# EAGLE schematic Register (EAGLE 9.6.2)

## Sheet 1 of 3: adressen
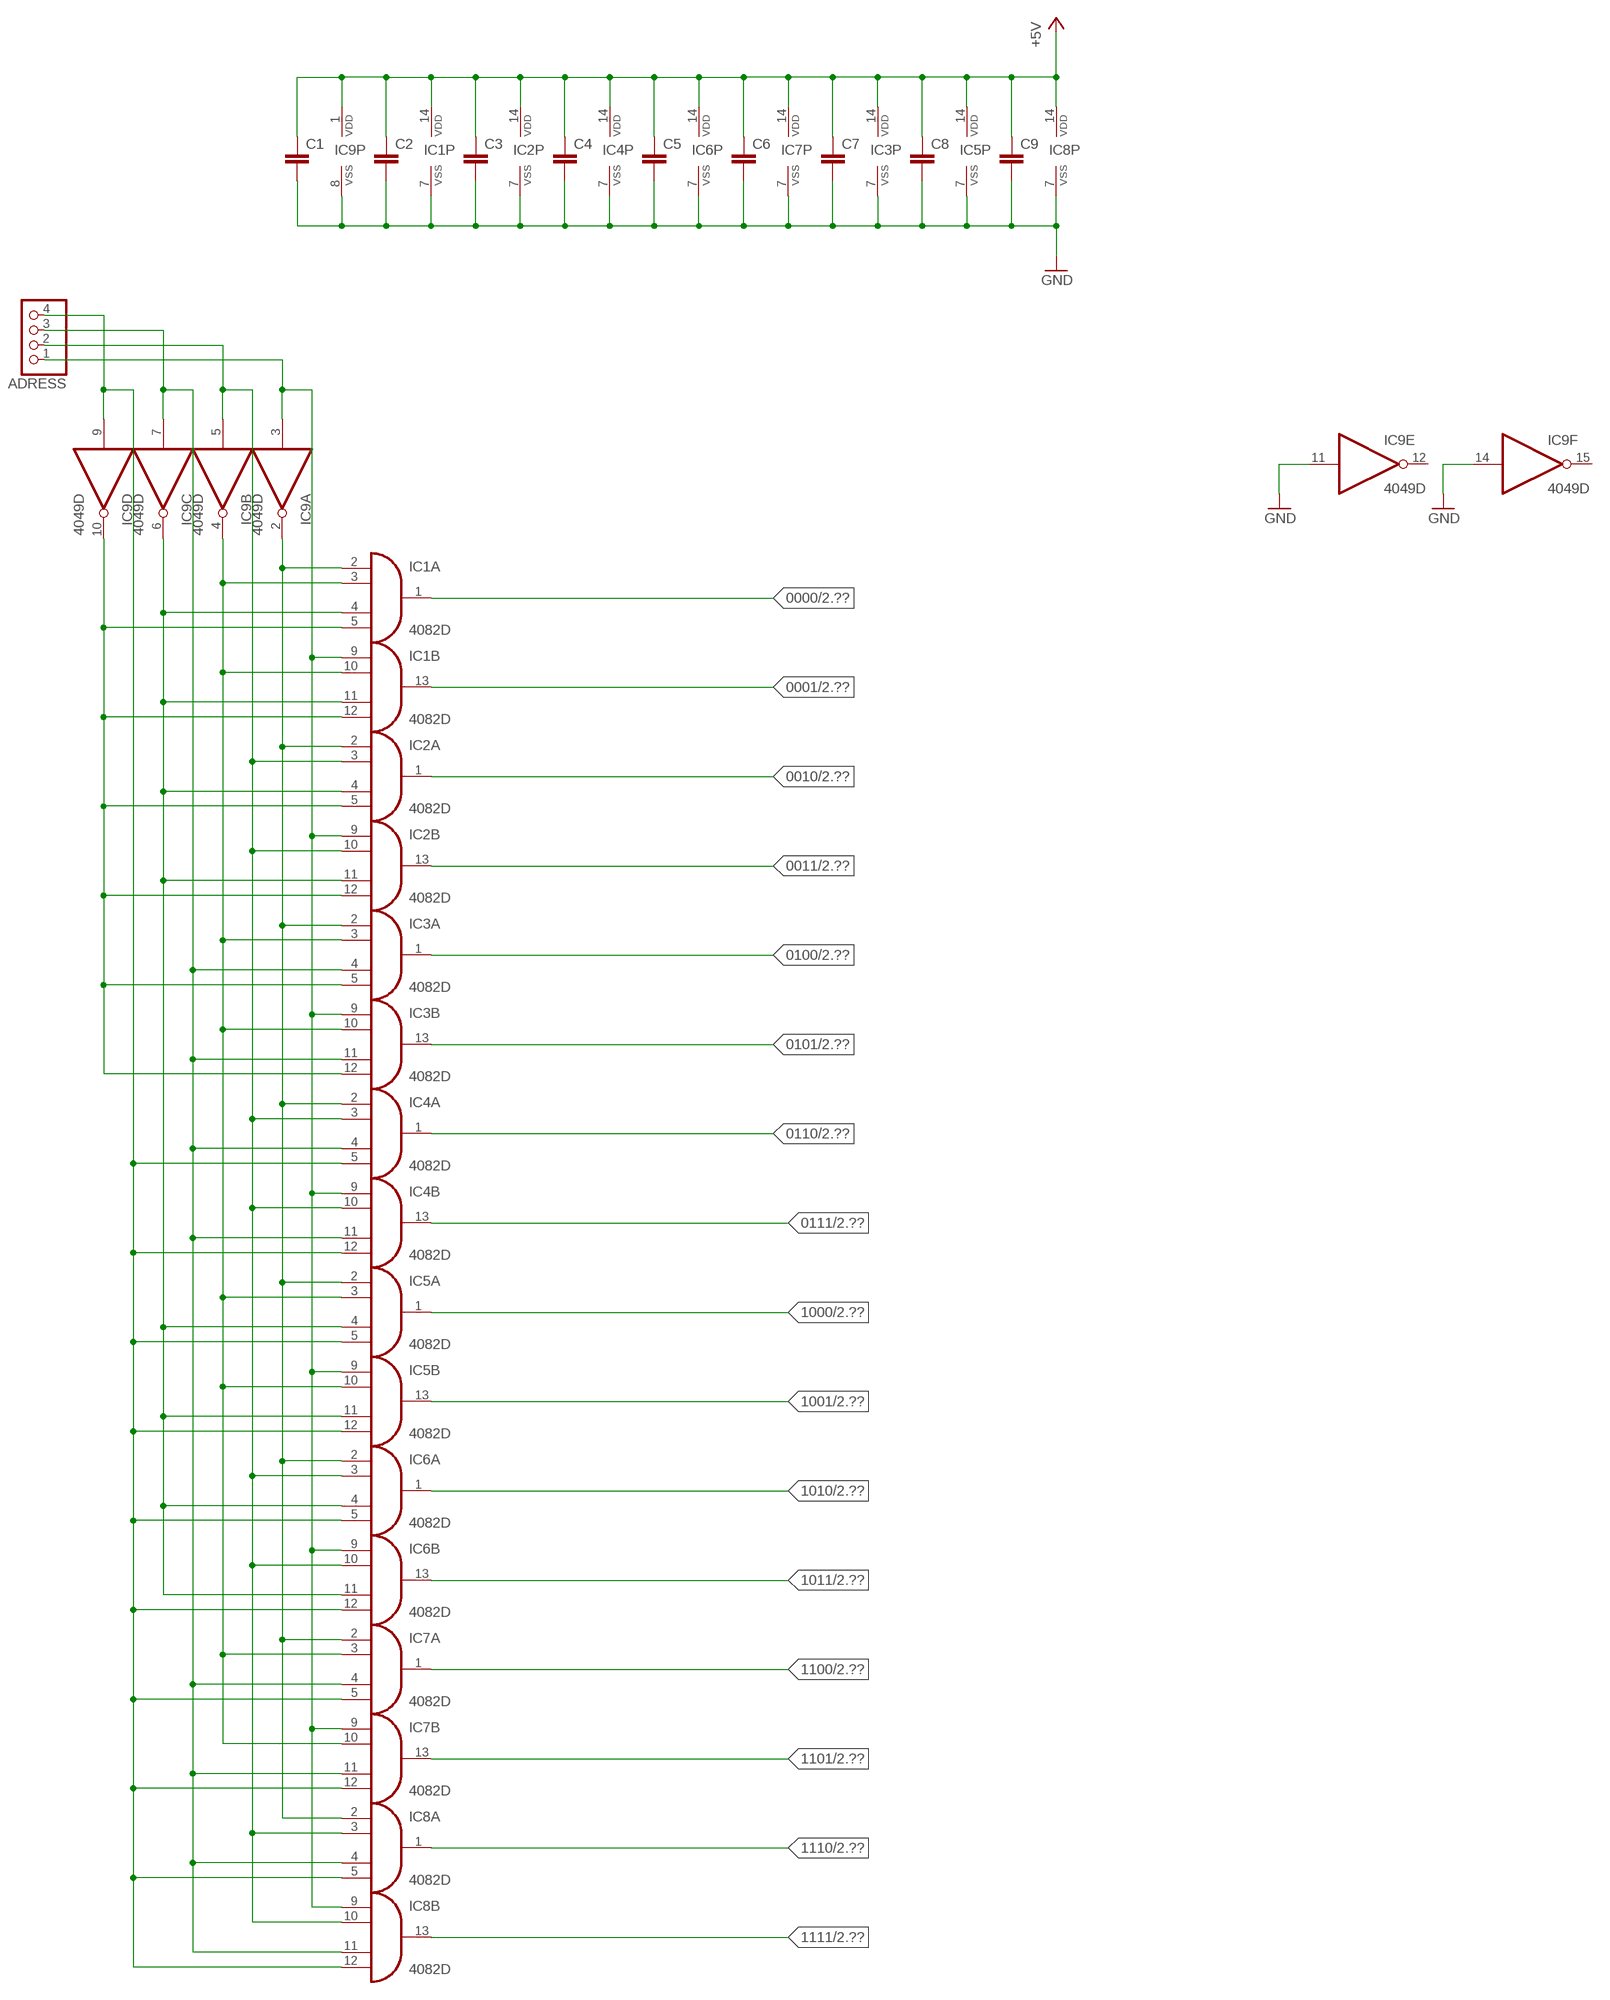
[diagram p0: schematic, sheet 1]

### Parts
ADRESS  PINHD-1X4  [1X04]
C1  C-EUC0805  [C0805]
C2  C-EUC0805  [C0805]
C3  C-EUC0805  [C0805]
C4  C-EUC0805  [C0805]
C5  C-EUC0805  [C0805]
C6  C-EUC0805  [C0805]
C7  C-EUC0805  [C0805]
C8  C-EUC0805  [C0805]
C9  C-EUC0805  [C0805]
IC1  4082D  [SO14]
IC2  4082D  [SO14]
IC3  4082D  [SO14]
IC4  4082D  [SO14]
IC5  4082D  [SO14]
IC6  4082D  [SO14]
IC7  4082D  [SO14]
IC8  4082D  [SO14]
IC9  4049D  [SO16]

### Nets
0000: IC1.1(A:O) ; also sheet 2
0001: IC1.13(B:O) ; also sheet 2
0010: IC2.1(A:O) ; also sheet 2
0011: IC2.13(B:O) ; also sheet 2
0100: IC3.1(A:O) ; also sheet 2
0101: IC3.13(B:O) ; also sheet 2
0110: IC4.1(A:O) ; also sheet 2
0111: IC4.13(B:O) ; also sheet 2
1000: IC5.1(A:O) ; also sheet 2
1001: IC5.13(B:O) ; also sheet 2
1010: IC6.1(A:O) ; also sheet 2
1011: IC6.13(B:O) ; also sheet 2
1100: IC7.1(A:O) ; also sheet 2
1101: IC7.13(B:O) ; also sheet 2
1110: IC8.1(A:O) ; also sheet 2
1111: IC8.13(B:O) ; also sheet 2
+5V: C1.1 C2.1 C3.1 C4.1 C5.1 C6.1 C7.1 C8.1 C9.1 IC1.14(P:VDD) IC2.14(P:VDD) IC3.14(P:VDD) IC4.14(P:VDD) IC5.14(P:VDD) IC6.14(P:VDD) IC7.14(P:VDD) IC8.14(P:VDD) IC9.1(P:VDD) ; also sheet 2,3
GND: C1.2 C2.2 C3.2 C4.2 C5.2 C6.2 C7.2 C8.2 C9.2 IC1.7(P:VSS) IC2.7(P:VSS) IC3.7(P:VSS) IC4.7(P:VSS) IC5.7(P:VSS) IC6.7(P:VSS) IC7.7(P:VSS) IC8.7(P:VSS) IC9.8(P:VSS) IC9.11(E:I) IC9.14(F:I) ; also sheet 2,3
N$1: ADRESS.1 IC1.9(B:I0) IC2.9(B:I0) IC3.9(B:I0) IC4.9(B:I0) IC5.9(B:I0) IC6.9(B:I0) IC7.9(B:I0) IC8.9(B:I0) IC9.3(A:I)
N$2: IC1.2(A:I0) IC2.2(A:I0) IC3.2(A:I0) IC4.2(A:I0) IC5.2(A:I0) IC6.2(A:I0) IC7.2(A:I0) IC8.2(A:I0) IC9.2(A:O)
N$3: ADRESS.2 IC2.3(A:I1) IC2.10(B:I1) IC4.3(A:I1) IC4.10(B:I1) IC6.3(A:I1) IC6.10(B:I1) IC8.3(A:I1) IC8.10(B:I1) IC9.5(B:I)
N$4: IC1.3(A:I1) IC1.10(B:I1) IC3.3(A:I1) IC3.10(B:I1) IC5.3(A:I1) IC5.10(B:I1) IC7.3(A:I1) IC7.10(B:I1) IC9.4(B:O)
N$5: ADRESS.3 IC3.4(A:I2) IC3.11(B:I2) IC4.4(A:I2) IC4.11(B:I2) IC7.4(A:I2) IC7.11(B:I2) IC8.4(A:I2) IC8.11(B:I2) IC9.7(C:I)
N$6: IC1.4(A:I2) IC1.11(B:I2) IC2.4(A:I2) IC2.11(B:I2) IC5.4(A:I2) IC5.11(B:I2) IC6.4(A:I2) IC6.11(B:I2) IC9.6(C:O)
N$7: ADRESS.4 IC4.5(A:I3) IC4.12(B:I3) IC5.5(A:I3) IC5.12(B:I3) IC6.5(A:I3) IC6.12(B:I3) IC7.5(A:I3) IC7.12(B:I3) IC8.5(A:I3) IC8.12(B:I3) IC9.9(D:I)
N$8: IC1.5(A:I3) IC1.12(B:I3) IC2.5(A:I3) IC2.12(B:I3) IC3.5(A:I3) IC3.12(B:I3) IC9.10(D:O)
Unconnected: IC9.12(E:O) IC9.15(F:O)

## Sheet 2 of 3: 4x4Speicher
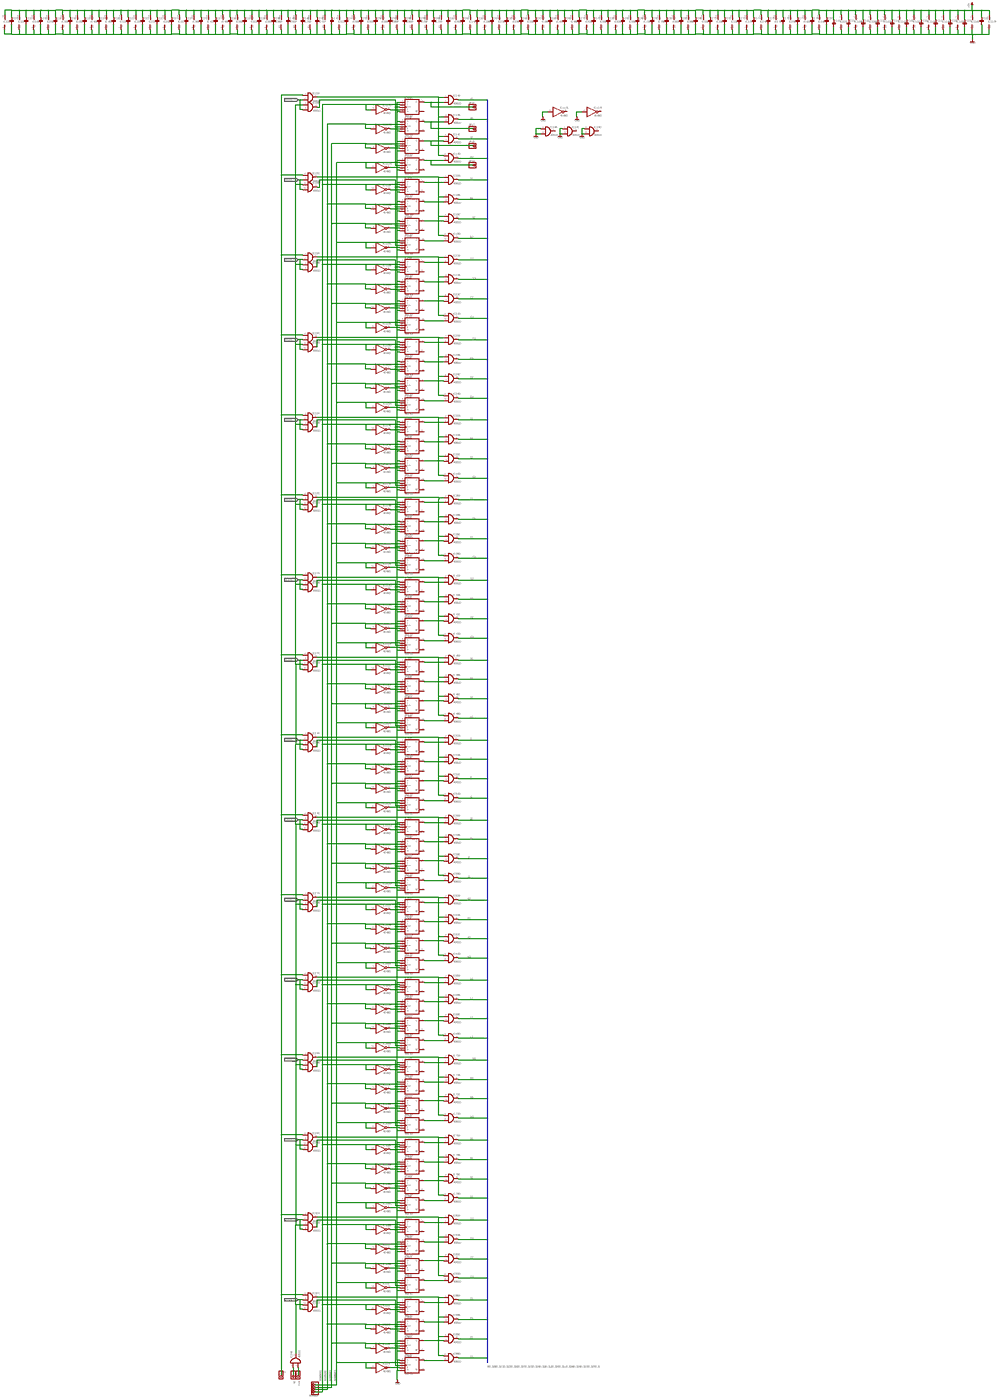
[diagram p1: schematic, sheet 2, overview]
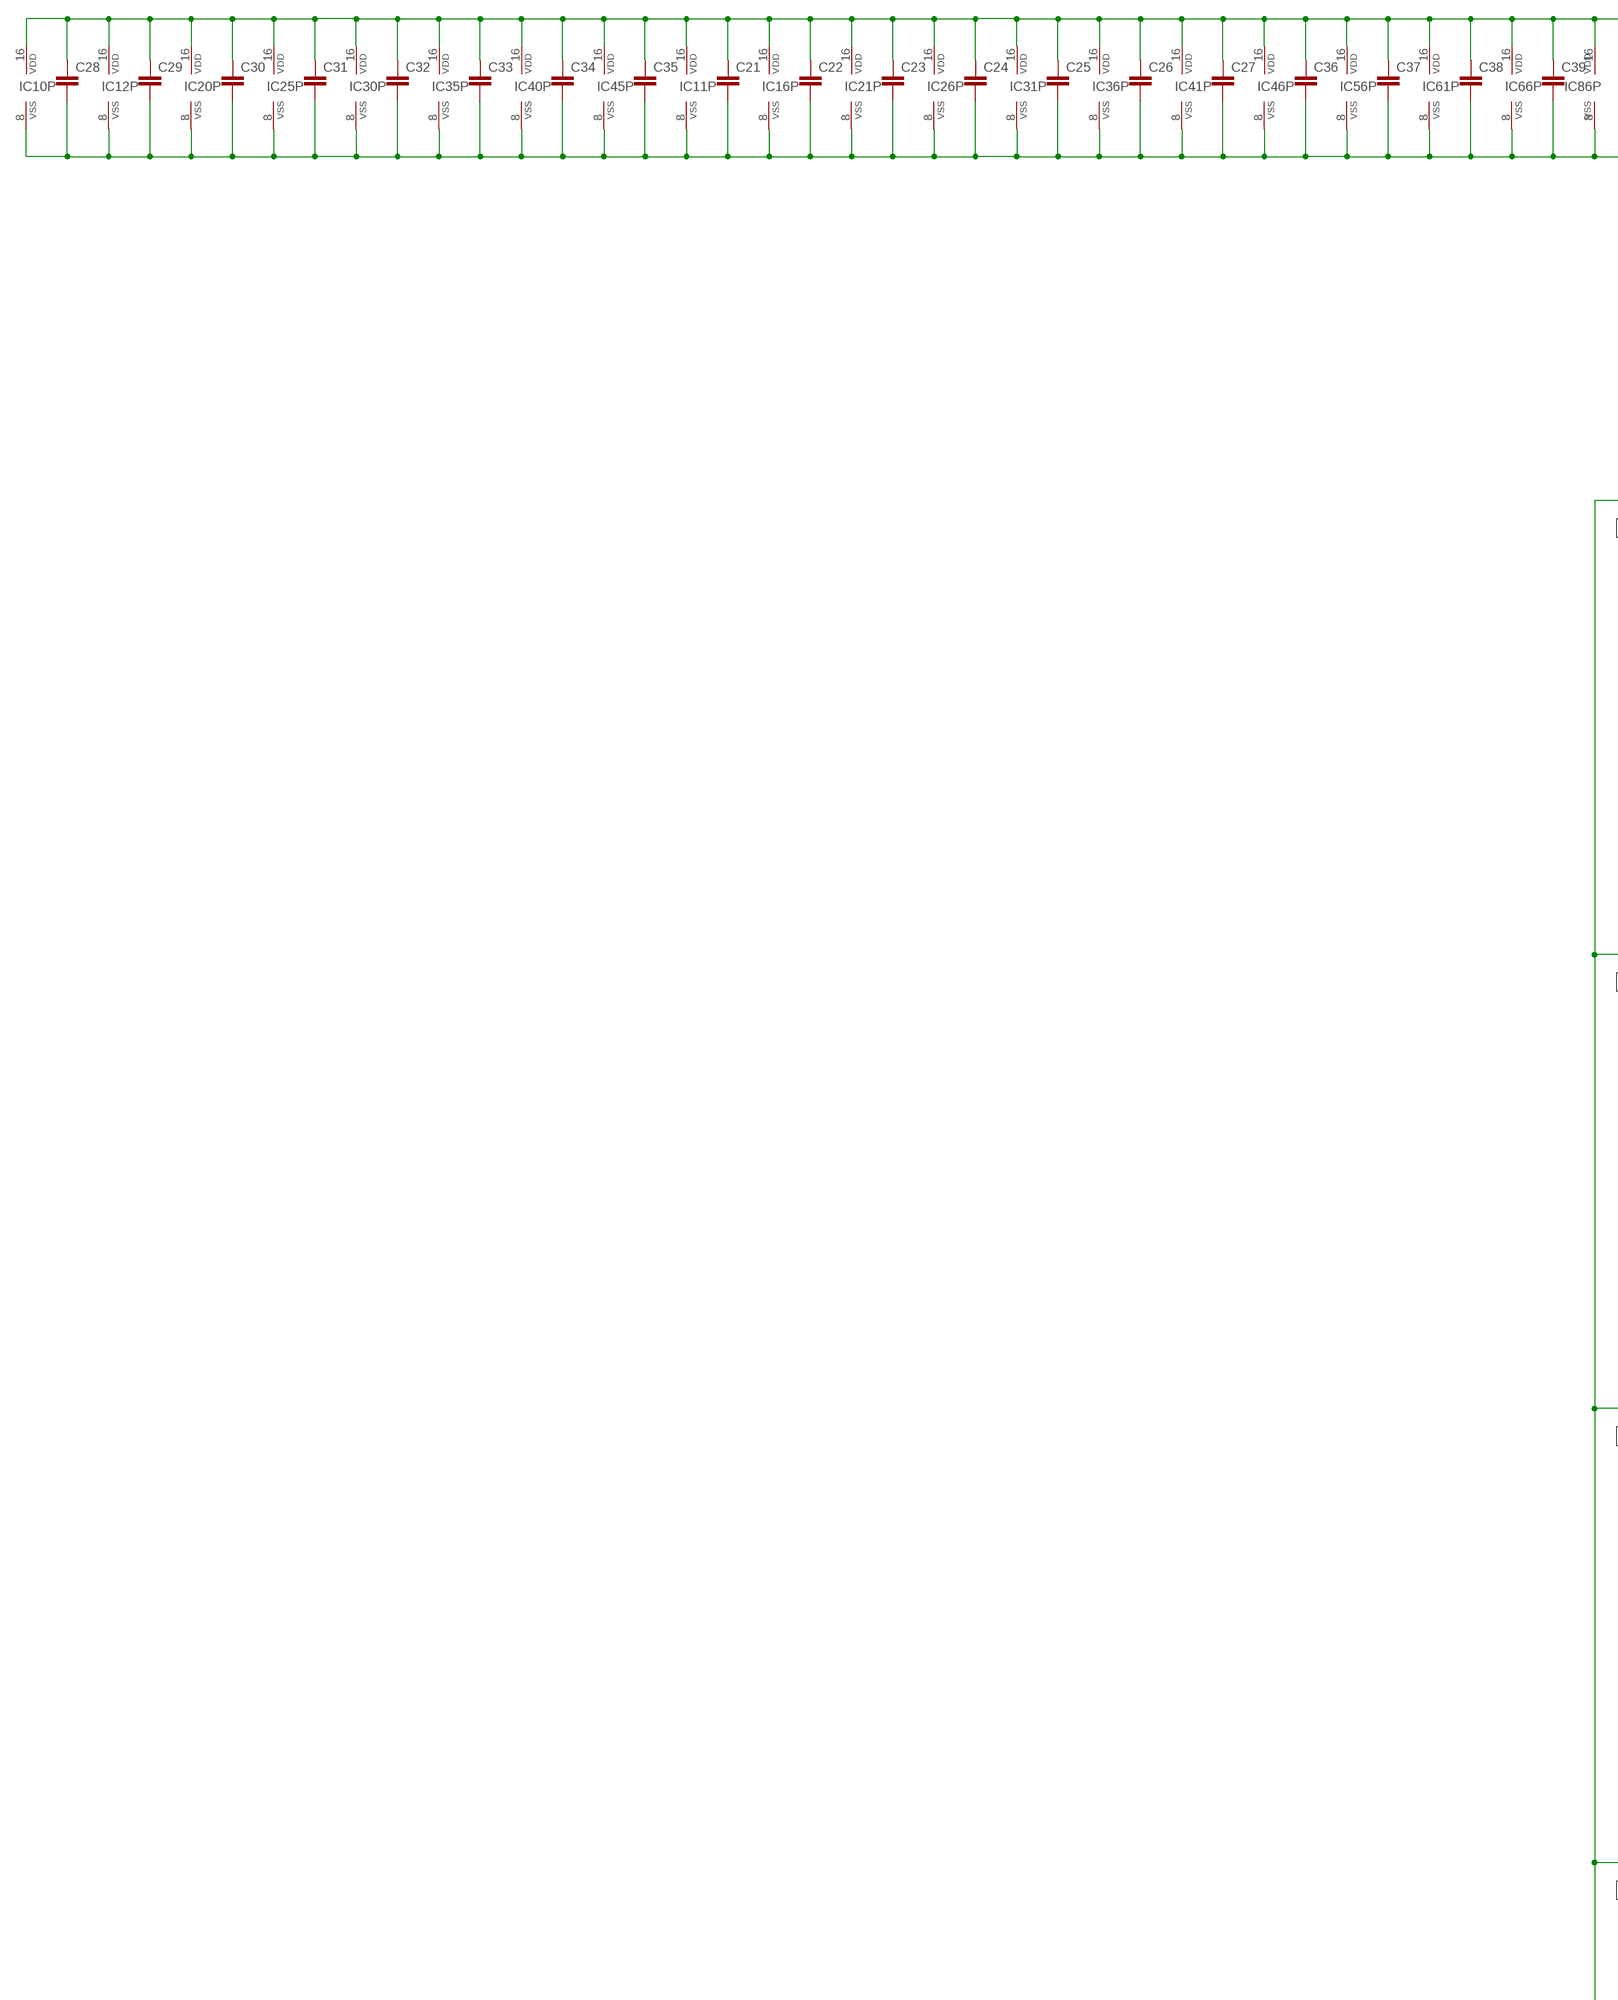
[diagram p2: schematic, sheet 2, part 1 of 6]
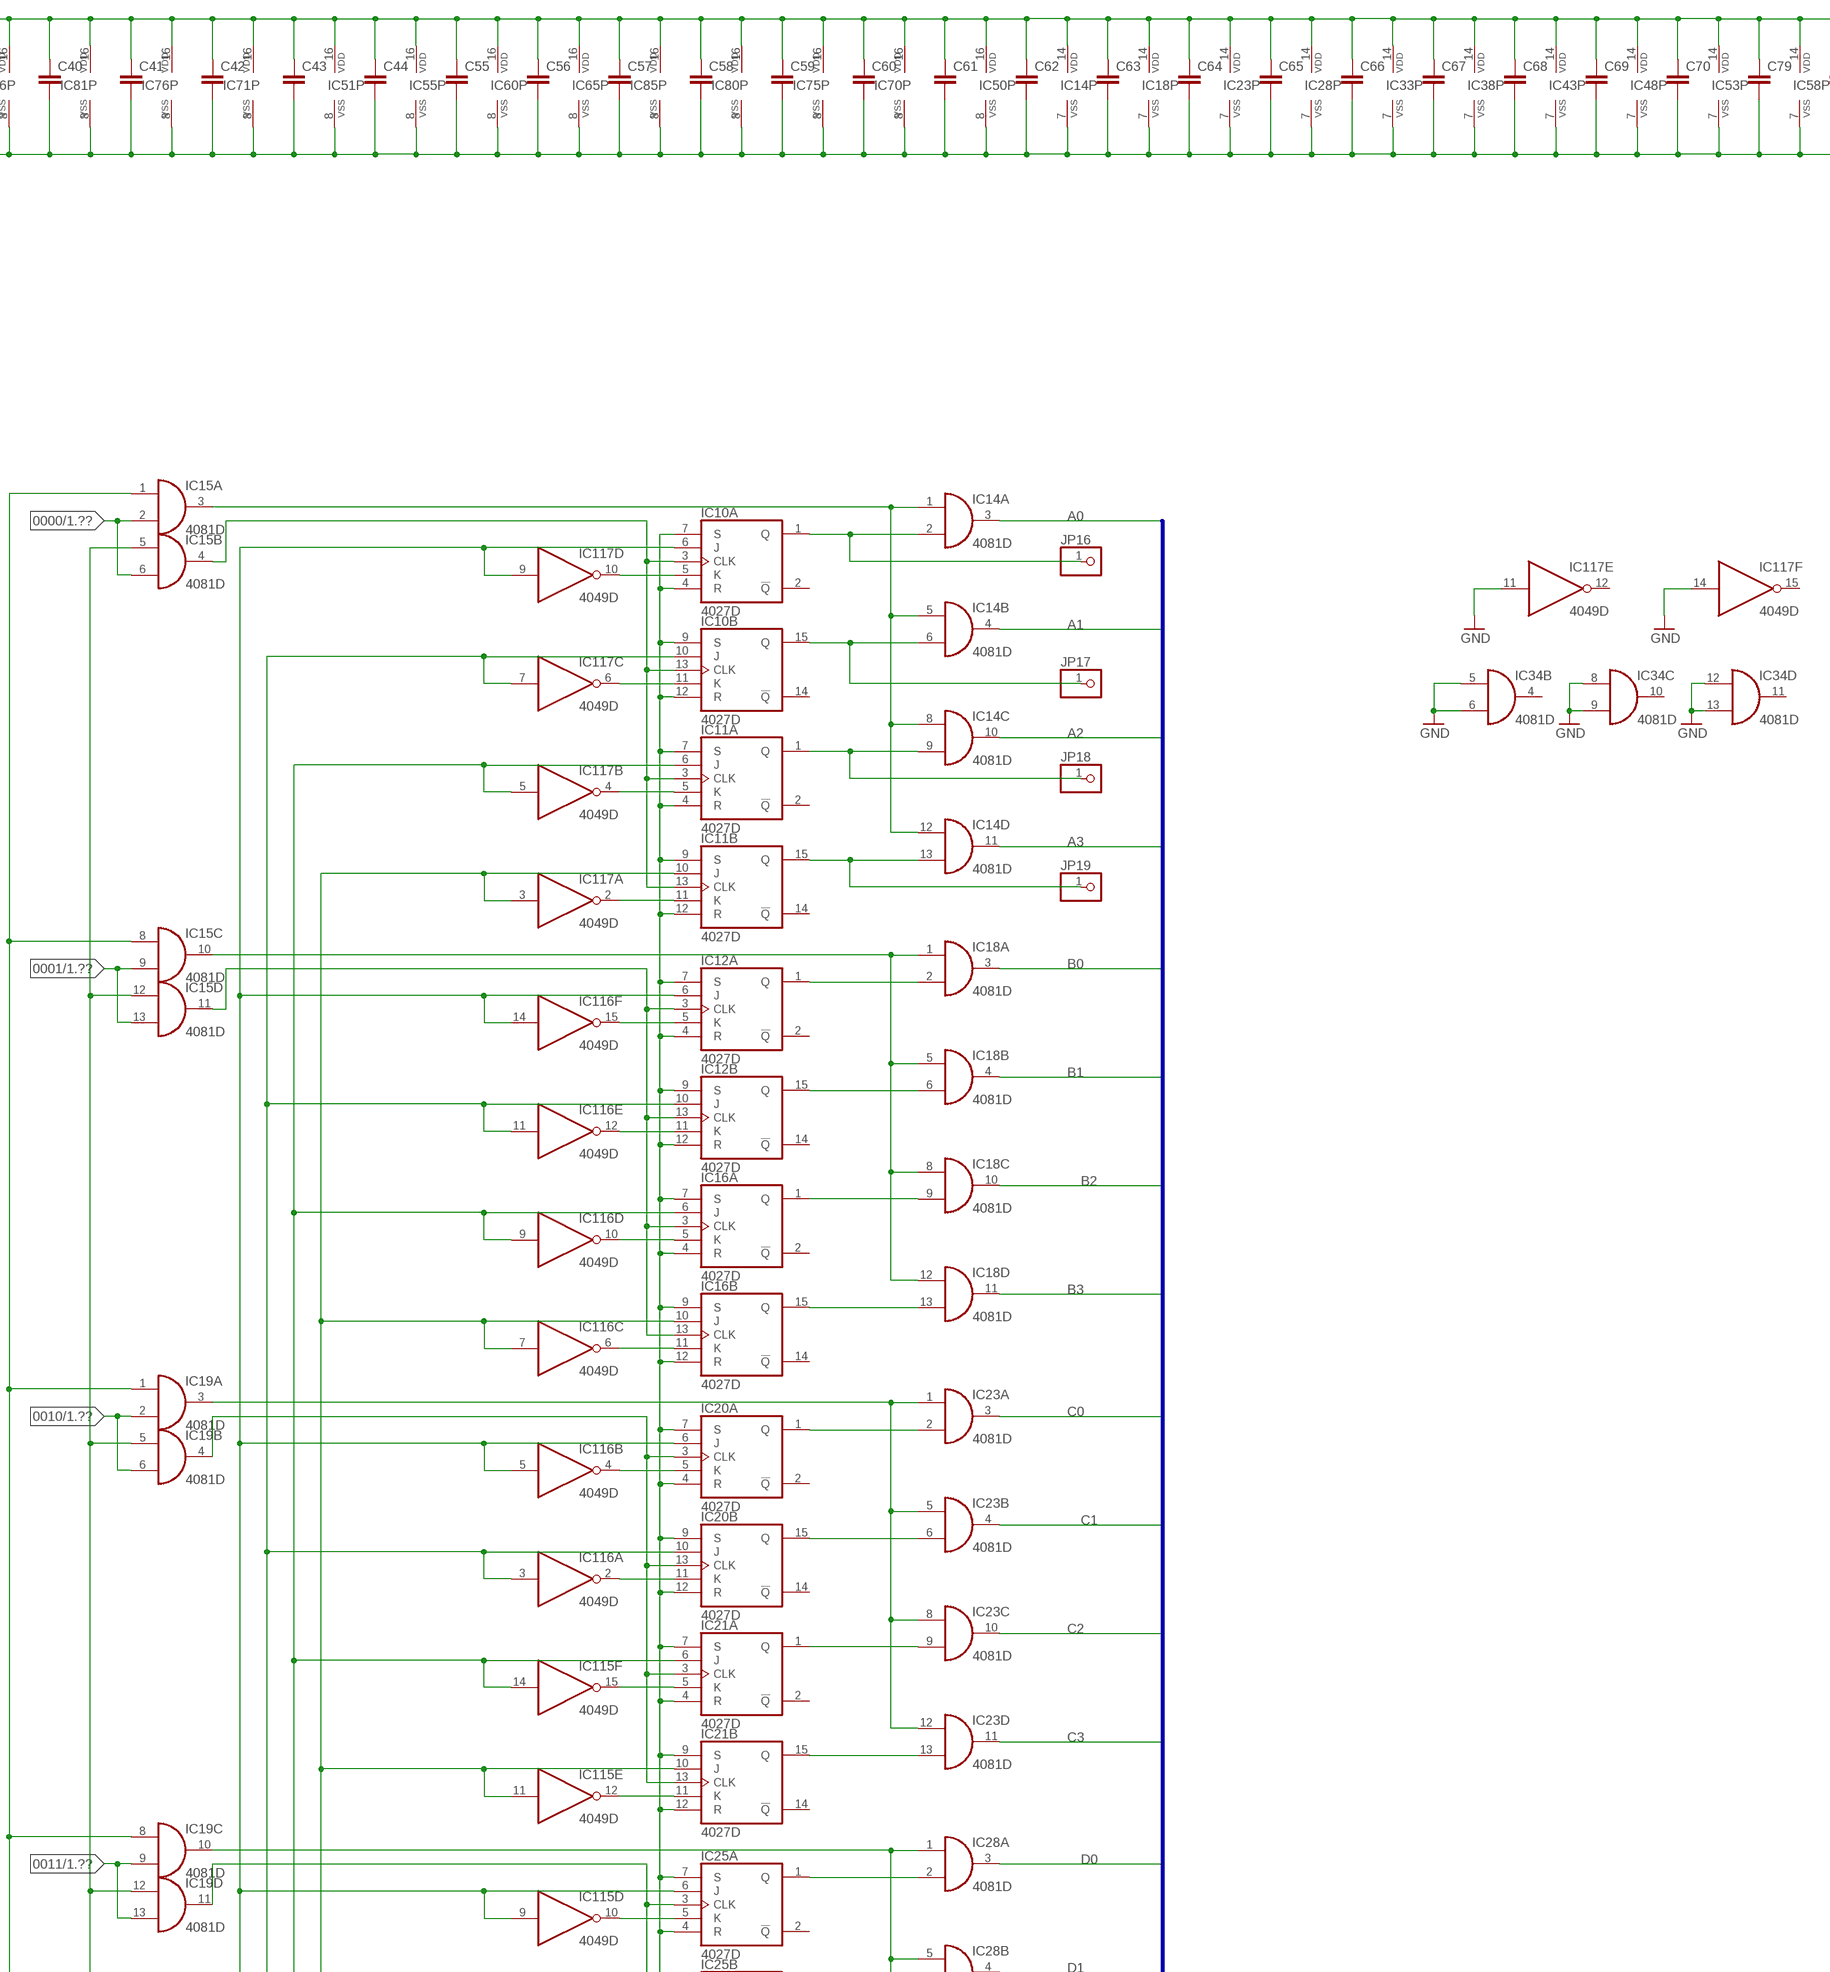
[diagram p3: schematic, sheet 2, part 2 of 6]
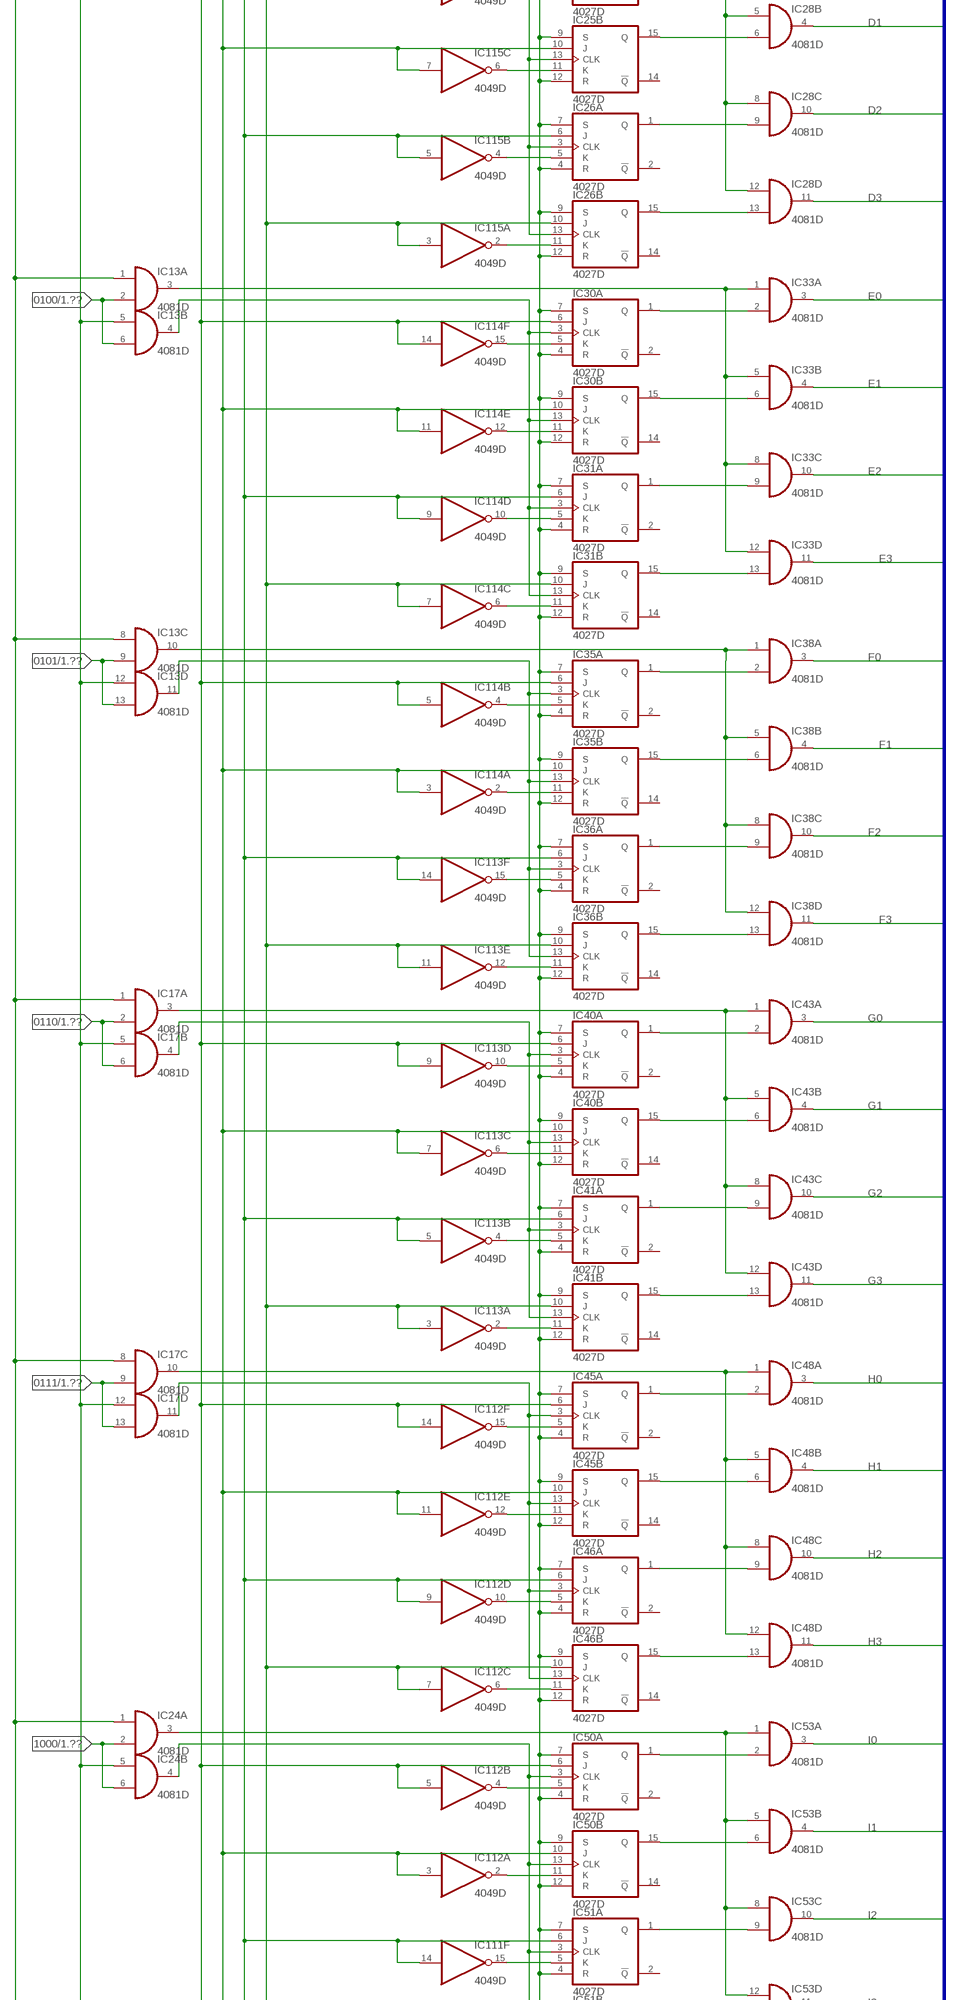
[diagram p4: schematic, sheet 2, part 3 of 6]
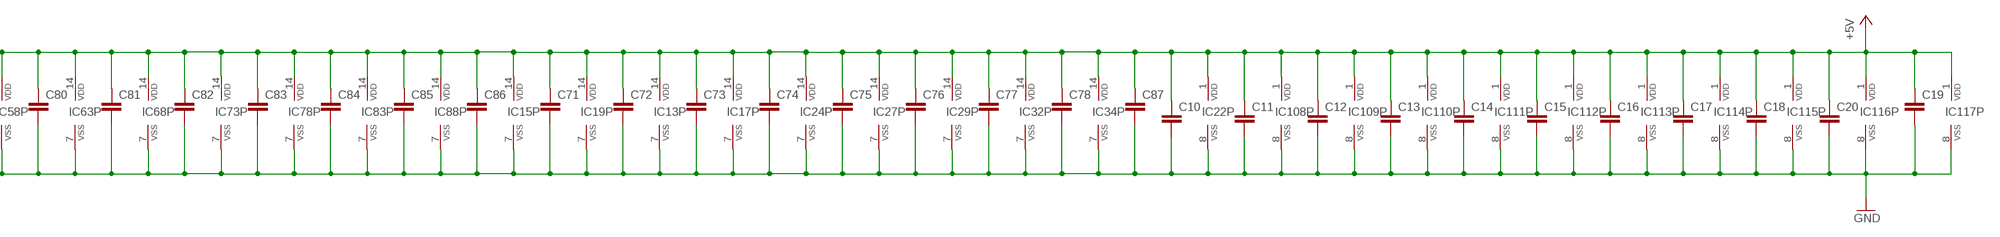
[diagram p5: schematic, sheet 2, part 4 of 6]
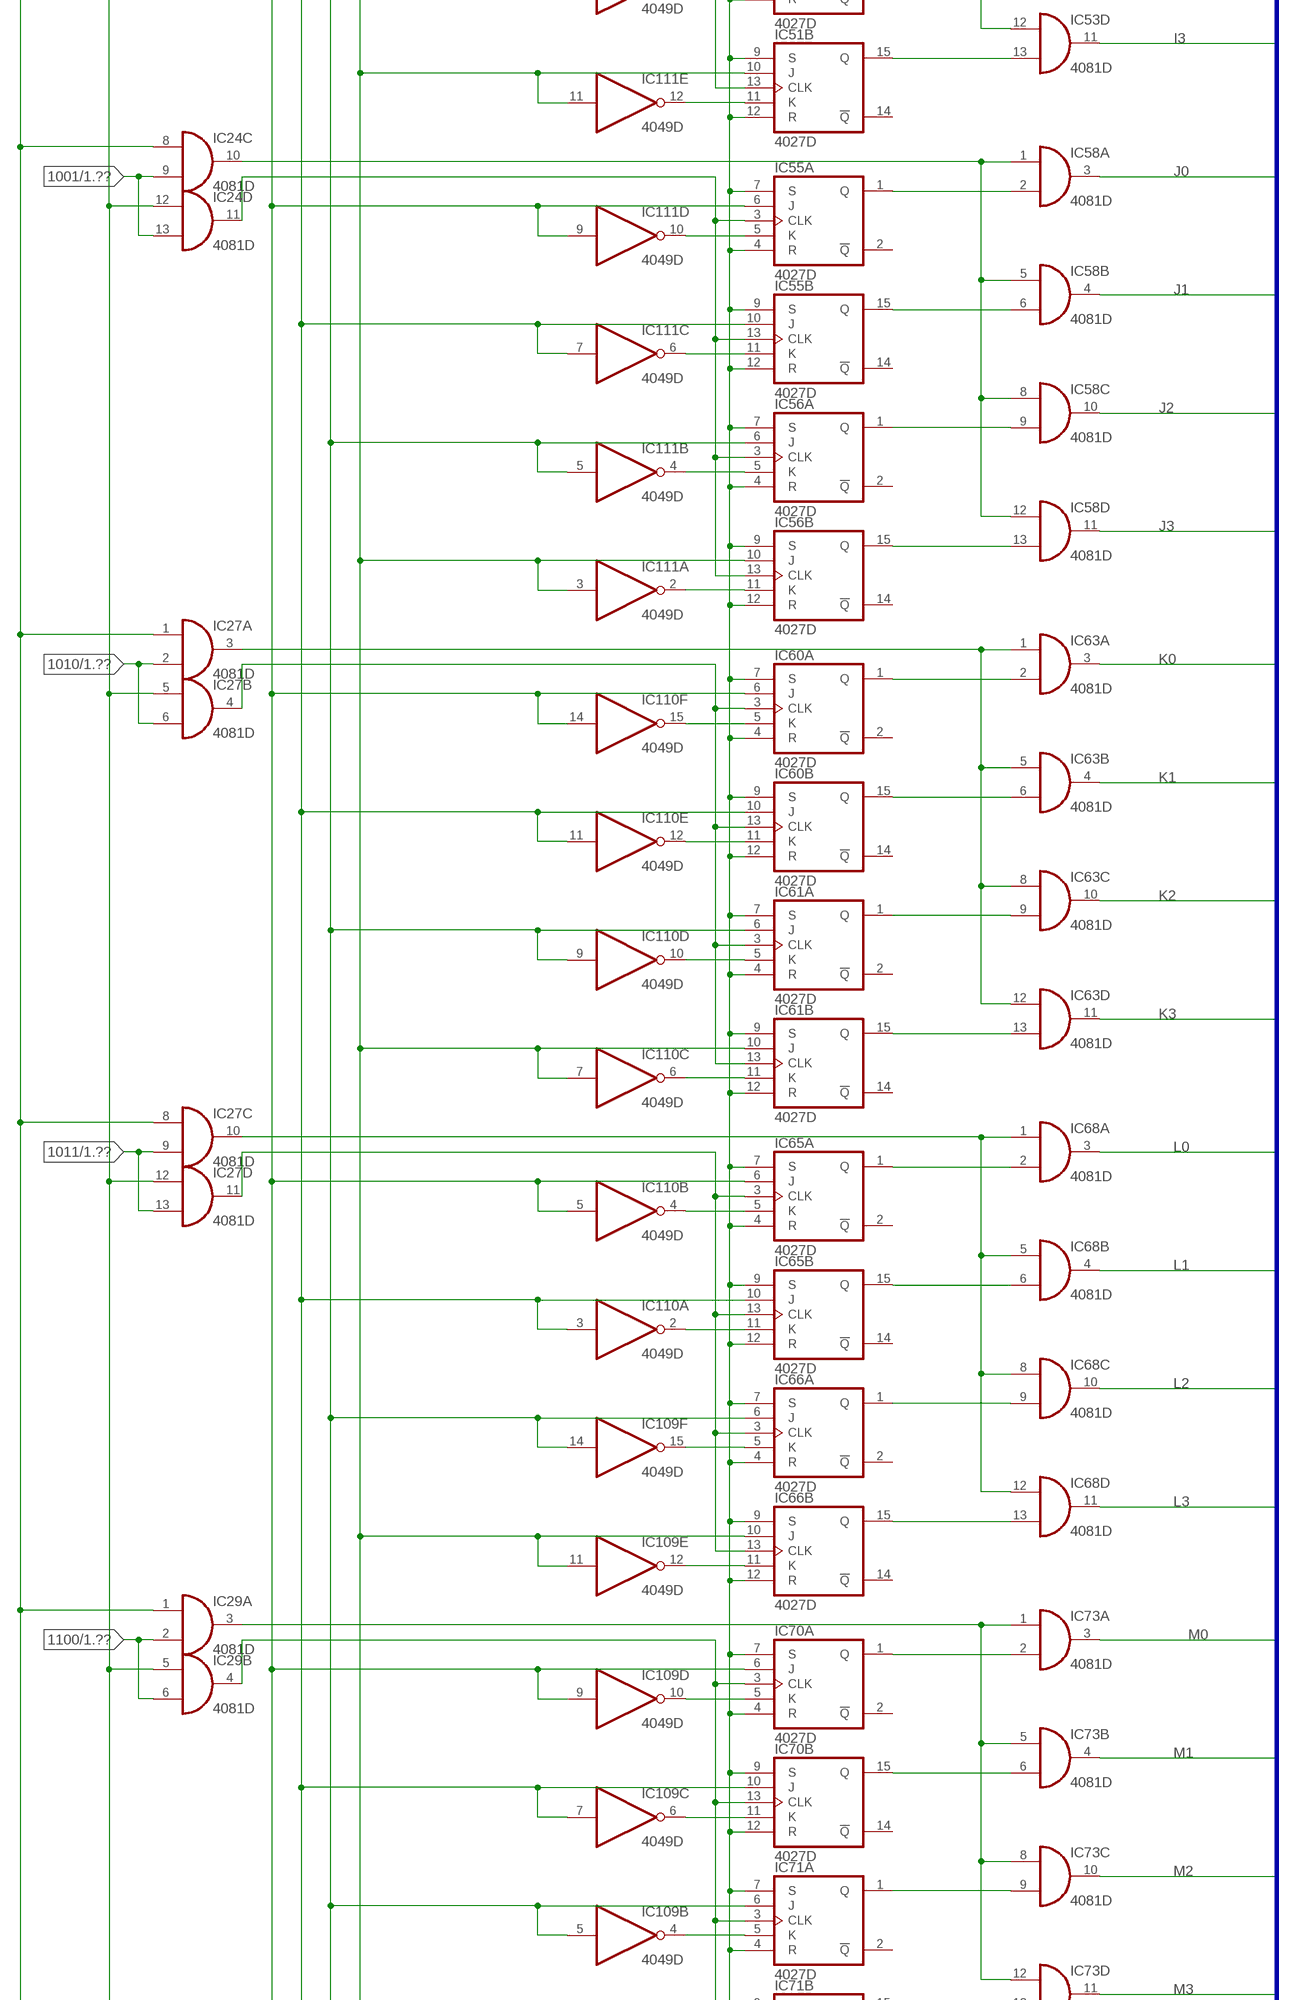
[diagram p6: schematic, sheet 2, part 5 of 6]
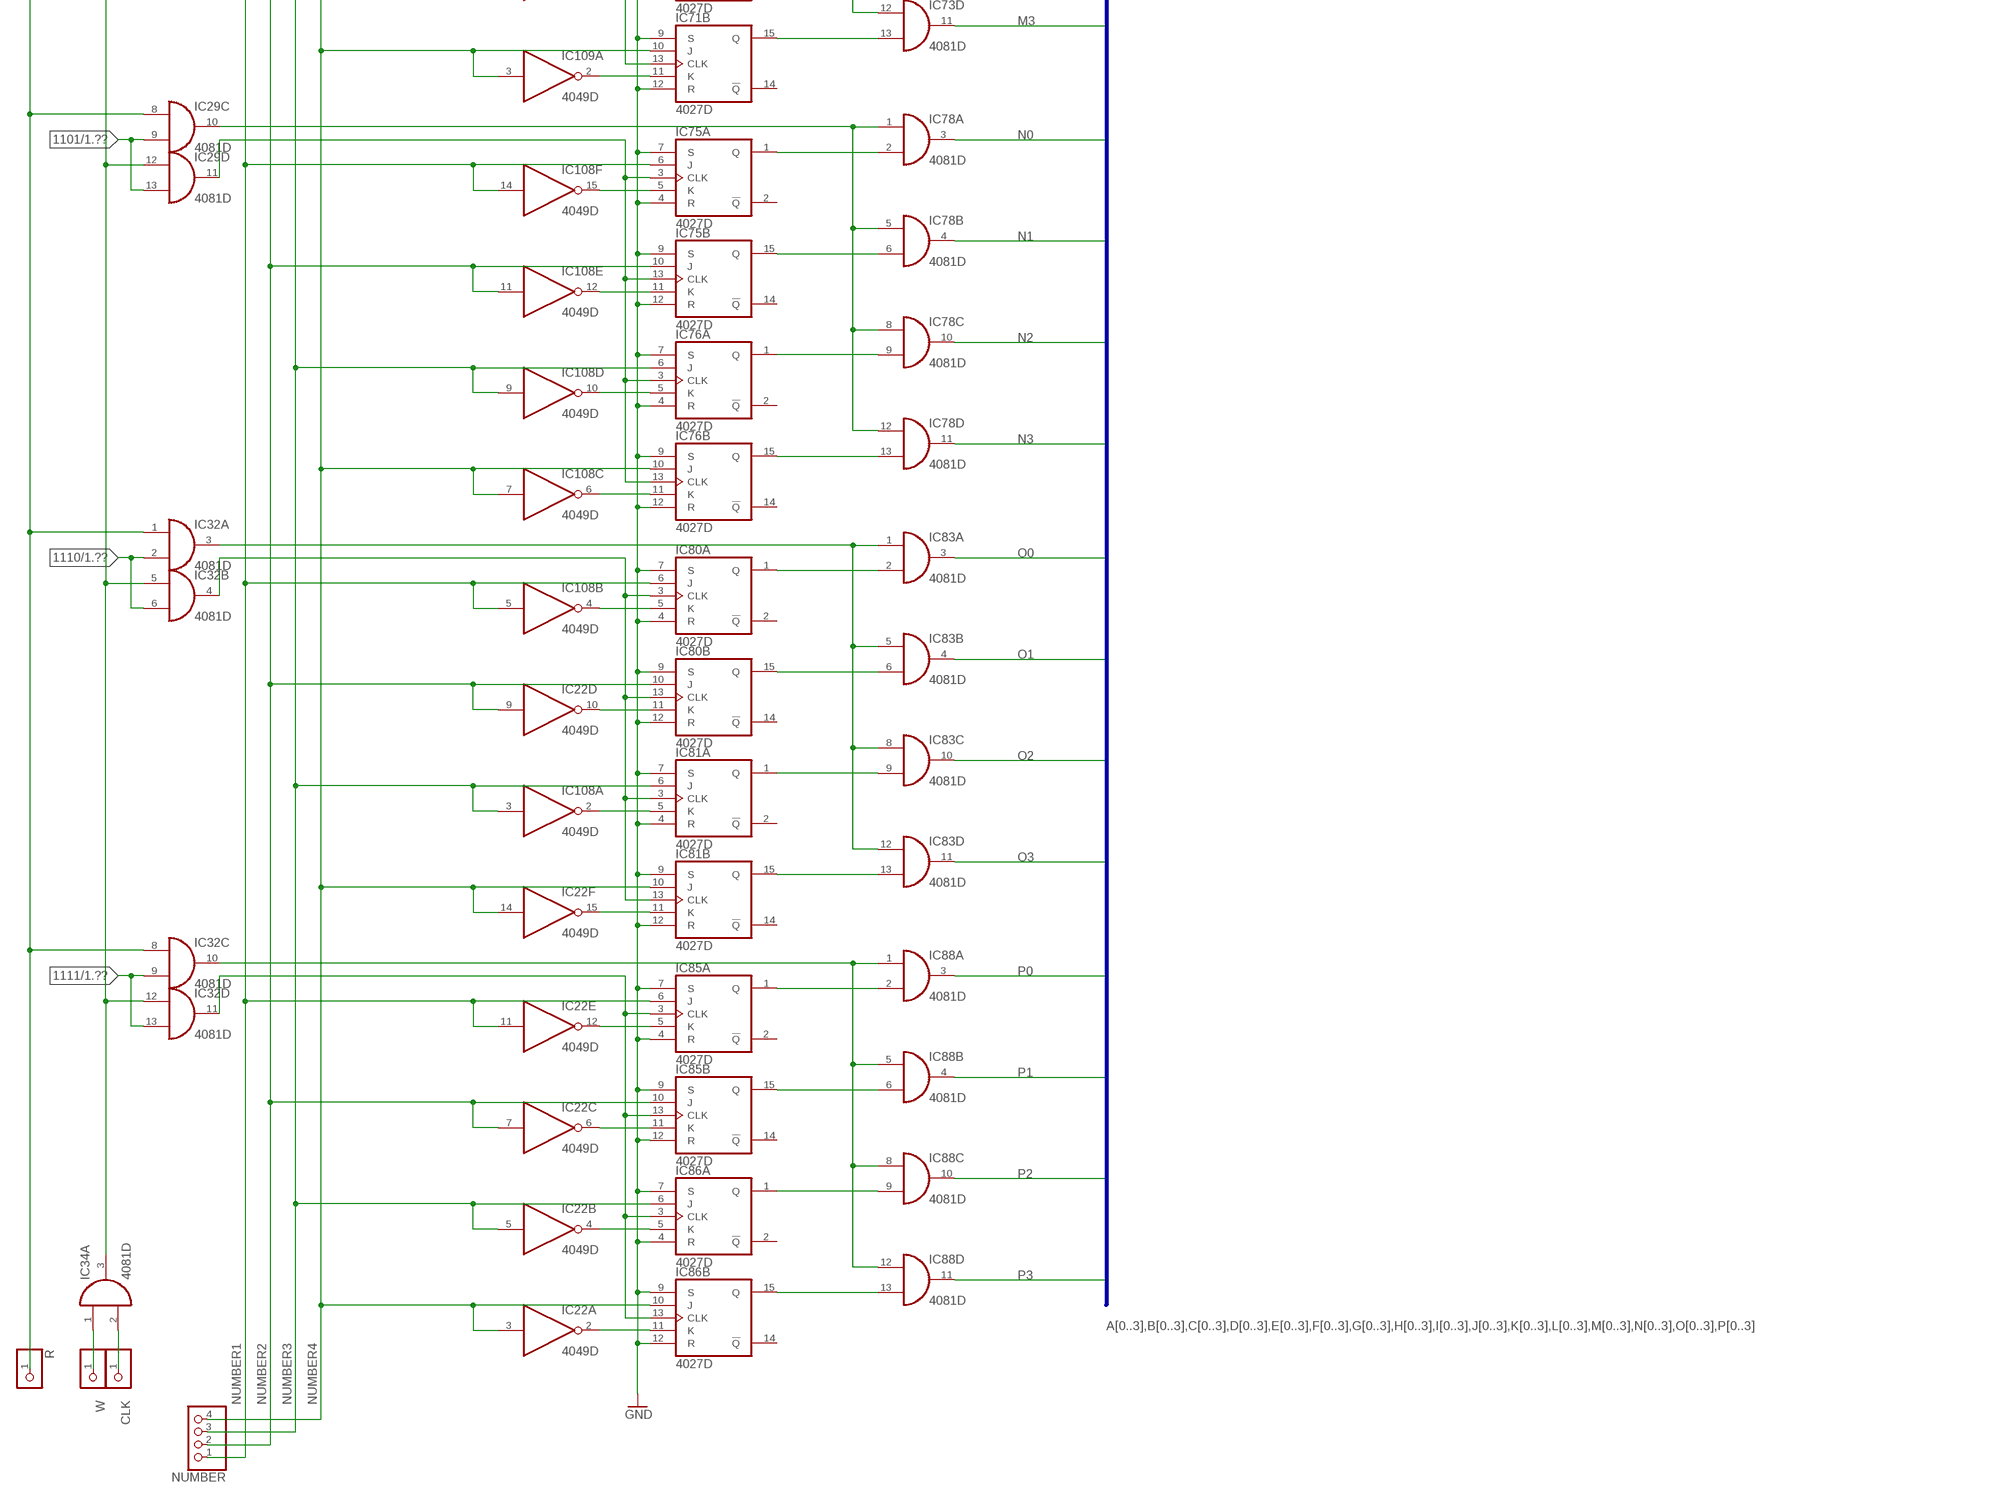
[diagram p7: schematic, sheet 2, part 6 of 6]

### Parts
C10  C-EUC0805  [C0805]
C11  C-EUC0805  [C0805]
C12  C-EUC0805  [C0805]
C13  C-EUC0805  [C0805]
C14  C-EUC0805  [C0805]
C15  C-EUC0805  [C0805]
C16  C-EUC0805  [C0805]
C17  C-EUC0805  [C0805]
C18  C-EUC0805  [C0805]
C19  C-EUC0805  [C0805]
C20  C-EUC0805  [C0805]
C21  C-EUC0805  [C0805]
C22  C-EUC0805  [C0805]
C23  C-EUC0805  [C0805]
C24  C-EUC0805  [C0805]
C25  C-EUC0805  [C0805]
C26  C-EUC0805  [C0805]
C27  C-EUC0805  [C0805]
C28  C-EUC0805  [C0805]
C29  C-EUC0805  [C0805]
C30  C-EUC0805  [C0805]
C31  C-EUC0805  [C0805]
C32  C-EUC0805  [C0805]
C33  C-EUC0805  [C0805]
C34  C-EUC0805  [C0805]
C35  C-EUC0805  [C0805]
C36  C-EUC0805  [C0805]
C37  C-EUC0805  [C0805]
C38  C-EUC0805  [C0805]
C39  C-EUC0805  [C0805]
C40  C-EUC0805  [C0805]
C41  C-EUC0805  [C0805]
C42  C-EUC0805  [C0805]
C43  C-EUC0805  [C0805]
C44  C-EUC0805  [C0805]
C55  C-EUC0805  [C0805]
C56  C-EUC0805  [C0805]
C57  C-EUC0805  [C0805]
C58  C-EUC0805  [C0805]
C59  C-EUC0805  [C0805]
C60  C-EUC0805  [C0805]
C61  C-EUC0805  [C0805]
C62  C-EUC0805  [C0805]
C63  C-EUC0805  [C0805]
C64  C-EUC0805  [C0805]
C65  C-EUC0805  [C0805]
C66  C-EUC0805  [C0805]
C67  C-EUC0805  [C0805]
C68  C-EUC0805  [C0805]
C69  C-EUC0805  [C0805]
C70  C-EUC0805  [C0805]
C71  C-EUC0805  [C0805]
C72  C-EUC0805  [C0805]
C73  C-EUC0805  [C0805]
C74  C-EUC0805  [C0805]
C75  C-EUC0805  [C0805]
C76  C-EUC0805  [C0805]
C77  C-EUC0805  [C0805]
C78  C-EUC0805  [C0805]
C79  C-EUC0805  [C0805]
C80  C-EUC0805  [C0805]
C81  C-EUC0805  [C0805]
C82  C-EUC0805  [C0805]
C83  C-EUC0805  [C0805]
C84  C-EUC0805  [C0805]
C85  C-EUC0805  [C0805]
C86  C-EUC0805  [C0805]
C87  C-EUC0805  [C0805]
CLK  PINHD-1X1  [1X01]
IC10  4027D  [SO16]
IC11  4027D  [SO16]
IC12  4027D  [SO16]
IC13  4081D  [SO14]
IC14  4081D  [SO14]
IC15  4081D  [SO14]
IC16  4027D  [SO16]
IC17  4081D  [SO14]
IC18  4081D  [SO14]
IC19  4081D  [SO14]
IC20  4027D  [SO16]
IC21  4027D  [SO16]
IC22  4049D  [SO16]
IC23  4081D  [SO14]
IC24  4081D  [SO14]
IC25  4027D  [SO16]
IC26  4027D  [SO16]
IC27  4081D  [SO14]
IC28  4081D  [SO14]
IC29  4081D  [SO14]
IC30  4027D  [SO16]
IC31  4027D  [SO16]
IC32  4081D  [SO14]
IC33  4081D  [SO14]
IC34  4081D  [SO14]
IC35  4027D  [SO16]
IC36  4027D  [SO16]
IC38  4081D  [SO14]
IC40  4027D  [SO16]
IC41  4027D  [SO16]
IC43  4081D  [SO14]
IC45  4027D  [SO16]
IC46  4027D  [SO16]
IC48  4081D  [SO14]
IC50  4027D  [SO16]
IC51  4027D  [SO16]
IC53  4081D  [SO14]
IC55  4027D  [SO16]
IC56  4027D  [SO16]
IC58  4081D  [SO14]
IC60  4027D  [SO16]
IC61  4027D  [SO16]
IC63  4081D  [SO14]
IC65  4027D  [SO16]
IC66  4027D  [SO16]
IC68  4081D  [SO14]
IC70  4027D  [SO16]
IC71  4027D  [SO16]
IC73  4081D  [SO14]
IC75  4027D  [SO16]
IC76  4027D  [SO16]
IC78  4081D  [SO14]
IC80  4027D  [SO16]
IC81  4027D  [SO16]
IC83  4081D  [SO14]
IC85  4027D  [SO16]
IC86  4027D  [SO16]
IC88  4081D  [SO14]
IC108  4049D  [SO16]
IC109  4049D  [SO16]
IC110  4049D  [SO16]
IC111  4049D  [SO16]
IC112  4049D  [SO16]
IC113  4049D  [SO16]
IC114  4049D  [SO16]
IC115  4049D  [SO16]
IC116  4049D  [SO16]
IC117  4049D  [SO16]
JP16  PINHD-1X1  [1X01]
JP17  PINHD-1X1  [1X01]
JP18  PINHD-1X1  [1X01]
JP19  PINHD-1X1  [1X01]
NUMBER  PINHD-1X4  [1X04]
R  PINHD-1X1  [1X01]
W  PINHD-1X1  [1X01]

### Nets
0000: IC15.2(A:I1) IC15.6(B:I1) ; also sheet 1
0001: IC15.9(C:I1) IC15.13(D:I1) ; also sheet 1
0010: IC19.2(A:I1) IC19.6(B:I1) ; also sheet 1
0011: IC19.9(C:I1) IC19.13(D:I1) ; also sheet 1
0100: IC13.2(A:I1) IC13.6(B:I1) ; also sheet 1
0101: IC13.9(C:I1) IC13.13(D:I1) ; also sheet 1
0110: IC17.2(A:I1) IC17.6(B:I1) ; also sheet 1
0111: IC17.9(C:I1) IC17.13(D:I1) ; also sheet 1
1000: IC24.2(A:I1) IC24.6(B:I1) ; also sheet 1
1001: IC24.9(C:I1) IC24.13(D:I1) ; also sheet 1
1010: IC27.2(A:I1) IC27.6(B:I1) ; also sheet 1
1011: IC27.9(C:I1) IC27.13(D:I1) ; also sheet 1
1100: IC29.2(A:I1) IC29.6(B:I1) ; also sheet 1
1101: IC29.9(C:I1) IC29.13(D:I1) ; also sheet 1
1110: IC32.2(A:I1) IC32.6(B:I1) ; also sheet 1
1111: IC32.9(C:I1) IC32.13(D:I1) ; also sheet 1
+5V: C10.1 C11.1 C12.1 C13.1 C14.1 C15.1 C16.1 C17.1 C18.1 C19.1 C20.1 C21.1 C22.1 C23.1 C24.1 C25.1 C26.1 C27.1 C28.1 C29.1 C30.1 C31.1 C32.1 C33.1 C34.1 C35.1 C36.1 C37.1 C38.1 C39.1 C40.1 C41.1 C42.1 C43.1 C44.1 C55.1 C56.1 C57.1 C58.1 C59.1 C60.1 C61.1 C62.1 C63.1 C64.1 C65.1 C66.1 C67.1 C68.1 C69.1 C70.1 C71.1 C72.1 C73.1 C74.1 C75.1 C76.1 C77.1 C78.1 C79.1 C80.1 C81.1 C82.1 C83.1 C84.1 C85.1 C86.1 C87.1 IC10.16(P:VDD) IC11.16(P:VDD) IC12.16(P:VDD) IC13.14(P:VDD) IC14.14(P:VDD) IC15.14(P:VDD) IC16.16(P:VDD) IC17.14(P:VDD) IC18.14(P:VDD) IC19.14(P:VDD) IC20.16(P:VDD) IC21.16(P:VDD) IC22.1(P:VDD) IC23.14(P:VDD) IC24.14(P:VDD) IC25.16(P:VDD) IC26.16(P:VDD) IC27.14(P:VDD) IC28.14(P:VDD) IC29.14(P:VDD) IC30.16(P:VDD) IC31.16(P:VDD) IC32.14(P:VDD) IC33.14(P:VDD) IC34.14(P:VDD) IC35.16(P:VDD) IC36.16(P:VDD) IC38.14(P:VDD) IC40.16(P:VDD) IC41.16(P:VDD) IC43.14(P:VDD) IC45.16(P:VDD) IC46.16(P:VDD) IC48.14(P:VDD) IC50.16(P:VDD) IC51.16(P:VDD) IC53.14(P:VDD) IC55.16(P:VDD) IC56.16(P:VDD) IC58.14(P:VDD) IC60.16(P:VDD) IC61.16(P:VDD) IC63.14(P:VDD) IC65.16(P:VDD) IC66.16(P:VDD) IC68.14(P:VDD) IC70.16(P:VDD) IC71.16(P:VDD) IC73.14(P:VDD) IC75.16(P:VDD) IC76.16(P:VDD) IC78.14(P:VDD) IC80.16(P:VDD) IC81.16(P:VDD) IC83.14(P:VDD) IC85.16(P:VDD) IC86.16(P:VDD) IC88.14(P:VDD) IC108.1(P:VDD) IC109.1(P:VDD) IC110.1(P:VDD) IC111.1(P:VDD) IC112.1(P:VDD) IC113.1(P:VDD) IC114.1(P:VDD) IC115.1(P:VDD) IC116.1(P:VDD) IC117.1(P:VDD) ; also sheet 1,3
A0: IC14.3(A:O) ; also sheet 3
A1: IC14.4(B:O) ; also sheet 3
A2: IC14.10(C:O) ; also sheet 3
A3: IC14.11(D:O) ; also sheet 3
B0: IC18.3(A:O) ; also sheet 3
B1: IC18.4(B:O) ; also sheet 3
B2: IC18.10(C:O) ; also sheet 3
B3: IC18.11(D:O) ; also sheet 3
C0: IC23.3(A:O) ; also sheet 3
C1: IC23.4(B:O) ; also sheet 3
C2: IC23.10(C:O) ; also sheet 3
C3: IC23.11(D:O) ; also sheet 3
D0: IC28.3(A:O) ; also sheet 3
D1: IC28.4(B:O) ; also sheet 3
D2: IC28.10(C:O) ; also sheet 3
D3: IC28.11(D:O) ; also sheet 3
E0: IC33.3(A:O) ; also sheet 3
E1: IC33.4(B:O) ; also sheet 3
E2: IC33.10(C:O) ; also sheet 3
E3: IC33.11(D:O) ; also sheet 3
F0: IC38.3(A:O) ; also sheet 3
F1: IC38.4(B:O) ; also sheet 3
F2: IC38.10(C:O) ; also sheet 3
F3: IC38.11(D:O) ; also sheet 3
G0: IC43.3(A:O) ; also sheet 3
G1: IC43.4(B:O) ; also sheet 3
G2: IC43.10(C:O) ; also sheet 3
G3: IC43.11(D:O) ; also sheet 3
GND: C10.2 C11.2 C12.2 C13.2 C14.2 C15.2 C16.2 C17.2 C18.2 C19.2 C20.2 C21.2 C22.2 C23.2 C24.2 C25.2 C26.2 C27.2 C28.2 C29.2 C30.2 C31.2 C32.2 C33.2 C34.2 C35.2 C36.2 C37.2 C38.2 C39.2 C40.2 C41.2 C42.2 C43.2 C44.2 C55.2 C56.2 C57.2 C58.2 C59.2 C60.2 C61.2 C62.2 C63.2 C64.2 C65.2 C66.2 C67.2 C68.2 C69.2 C70.2 C71.2 C72.2 C73.2 C74.2 C75.2 C76.2 C77.2 C78.2 C79.2 C80.2 C81.2 C82.2 C83.2 C84.2 C85.2 C86.2 C87.2 IC10.4(A:R) IC10.7(A:S) IC10.8(P:VSS) IC10.9(B:S) IC10.12(B:R) IC11.4(A:R) IC11.7(A:S) IC11.8(P:VSS) IC11.9(B:S) IC11.12(B:R) IC12.4(A:R) IC12.7(A:S) IC12.8(P:VSS) IC12.9(B:S) IC12.12(B:R) IC13.7(P:VSS) IC14.7(P:VSS) IC15.7(P:VSS) IC16.4(A:R) IC16.7(A:S) IC16.8(P:VSS) IC16.9(B:S) IC16.12(B:R) IC17.7(P:VSS) IC18.7(P:VSS) IC19.7(P:VSS) IC20.4(A:R) IC20.7(A:S) IC20.8(P:VSS) IC20.9(B:S) IC20.12(B:R) IC21.4(A:R) IC21.7(A:S) IC21.8(P:VSS) IC21.9(B:S) IC21.12(B:R) IC22.8(P:VSS) IC23.7(P:VSS) IC24.7(P:VSS) IC25.4(A:R) IC25.7(A:S) IC25.8(P:VSS) IC25.9(B:S) IC25.12(B:R) IC26.4(A:R) IC26.7(A:S) IC26.8(P:VSS) IC26.9(B:S) IC26.12(B:R) IC27.7(P:VSS) IC28.7(P:VSS) IC29.7(P:VSS) IC30.4(A:R) IC30.7(A:S) IC30.8(P:VSS) IC30.9(B:S) IC30.12(B:R) IC31.4(A:R) IC31.7(A:S) IC31.8(P:VSS) IC31.9(B:S) IC31.12(B:R) IC32.7(P:VSS) IC33.7(P:VSS) IC34.5(B:I0) IC34.6(B:I1) IC34.7(P:VSS) IC34.8(C:I0) IC34.9(C:I1) IC34.12(D:I0) IC34.13(D:I1) IC35.4(A:R) IC35.7(A:S) IC35.8(P:VSS) IC35.9(B:S) IC35.12(B:R) IC36.4(A:R) IC36.7(A:S) IC36.8(P:VSS) IC36.9(B:S) IC36.12(B:R) IC38.7(P:VSS) IC40.4(A:R) IC40.7(A:S) IC40.8(P:VSS) IC40.9(B:S) IC40.12(B:R) IC41.4(A:R) IC41.7(A:S) IC41.8(P:VSS) IC41.9(B:S) IC41.12(B:R) IC43.7(P:VSS) IC45.4(A:R) IC45.7(A:S) IC45.8(P:VSS) IC45.9(B:S) IC45.12(B:R) IC46.4(A:R) IC46.7(A:S) IC46.8(P:VSS) IC46.9(B:S) IC46.12(B:R) IC48.7(P:VSS) IC50.4(A:R) IC50.7(A:S) IC50.8(P:VSS) IC50.9(B:S) IC50.12(B:R) IC51.4(A:R) IC51.7(A:S) IC51.8(P:VSS) IC51.9(B:S) IC51.12(B:R) IC53.7(P:VSS) IC55.4(A:R) IC55.7(A:S) IC55.8(P:VSS) IC55.9(B:S) IC55.12(B:R) IC56.4(A:R) IC56.7(A:S) IC56.8(P:VSS) IC56.9(B:S) IC56.12(B:R) IC58.7(P:VSS) IC60.4(A:R) IC60.7(A:S) IC60.8(P:VSS) IC60.9(B:S) IC60.12(B:R) IC61.4(A:R) IC61.7(A:S) IC61.8(P:VSS) IC61.9(B:S) IC61.12(B:R) IC63.7(P:VSS) IC65.4(A:R) IC65.7(A:S) IC65.8(P:VSS) IC65.9(B:S) IC65.12(B:R) IC66.4(A:R) IC66.7(A:S) IC66.8(P:VSS) IC66.9(B:S) IC66.12(B:R) IC68.7(P:VSS) IC70.4(A:R) IC70.7(A:S) IC70.8(P:VSS) IC70.9(B:S) IC70.12(B:R) IC71.4(A:R) IC71.7(A:S) IC71.8(P:VSS) IC71.9(B:S) IC71.12(B:R) IC73.7(P:VSS) IC75.4(A:R) IC75.7(A:S) IC75.8(P:VSS) IC75.9(B:S) IC75.12(B:R) IC76.4(A:R) IC76.7(A:S) IC76.8(P:VSS) IC76.9(B:S) IC76.12(B:R) IC78.7(P:VSS) IC80.4(A:R) IC80.7(A:S) IC80.8(P:VSS) IC80.9(B:S) IC80.12(B:R) IC81.4(A:R) IC81.7(A:S) IC81.8(P:VSS) IC81.9(B:S) IC81.12(B:R) IC83.7(P:VSS) IC85.4(A:R) IC85.7(A:S) IC85.8(P:VSS) IC85.9(B:S) IC85.12(B:R) IC86.4(A:R) IC86.7(A:S) IC86.8(P:VSS) IC86.9(B:S) IC86.12(B:R) IC88.7(P:VSS) IC108.8(P:VSS) IC109.8(P:VSS) IC110.8(P:VSS) IC111.8(P:VSS) IC112.8(P:VSS) IC113.8(P:VSS) IC114.8(P:VSS) IC115.8(P:VSS) IC116.8(P:VSS) IC117.8(P:VSS) IC117.11(E:I) IC117.14(F:I) ; also sheet 1,3
H0: IC48.3(A:O) ; also sheet 3
H1: IC48.4(B:O) ; also sheet 3
H2: IC48.10(C:O) ; also sheet 3
H3: IC48.11(D:O) ; also sheet 3
I0: IC53.3(A:O) ; also sheet 3
I1: IC53.4(B:O) ; also sheet 3
I2: IC53.10(C:O) ; also sheet 3
I3: IC53.11(D:O) ; also sheet 3
J0: IC58.3(A:O) ; also sheet 3
J1: IC58.4(B:O) ; also sheet 3
J2: IC58.10(C:O) ; also sheet 3
J3: IC58.11(D:O) ; also sheet 3
K0: IC63.3(A:O) ; also sheet 3
K1: IC63.4(B:O) ; also sheet 3
K2: IC63.10(C:O) ; also sheet 3
K3: IC63.11(D:O) ; also sheet 3
L0: IC68.3(A:O) ; also sheet 3
L1: IC68.4(B:O) ; also sheet 3
L2: IC68.10(C:O) ; also sheet 3
L3: IC68.11(D:O) ; also sheet 3
M0: IC73.3(A:O) ; also sheet 3
M1: IC73.4(B:O) ; also sheet 3
M2: IC73.10(C:O) ; also sheet 3
M3: IC73.11(D:O) ; also sheet 3
N0: IC78.3(A:O) ; also sheet 3
N1: IC78.4(B:O) ; also sheet 3
N2: IC78.10(C:O) ; also sheet 3
N3: IC78.11(D:O) ; also sheet 3
N$9: IC32.10(C:O) IC88.1(A:I0) IC88.5(B:I0) IC88.8(C:I0) IC88.12(D:I0)
N$10: IC32.3(A:O) IC83.1(A:I0) IC83.5(B:I0) IC83.8(C:I0) IC83.12(D:I0)
N$11: IC29.10(C:O) IC78.1(A:I0) IC78.5(B:I0) IC78.8(C:I0) IC78.12(D:I0)
N$12: IC29.3(A:O) IC73.1(A:I0) IC73.5(B:I0) IC73.8(C:I0) IC73.12(D:I0)
N$13: IC12.3(A:CLK) IC12.13(B:CLK) IC15.11(D:O) IC16.3(A:CLK) IC16.13(B:CLK)
N$14: IC11.11(B:K) IC117.2(A:O)
N$15: IC11.5(A:K) IC117.4(B:O)
N$16: IC10.11(B:K) IC117.6(C:O)
N$17: IC10.5(A:K) IC117.10(D:O)
N$18: IC14.1(A:I0) IC14.5(B:I0) IC14.8(C:I0) IC14.12(D:I0) IC15.3(A:O)
N$19: IC19.10(C:O) IC28.1(A:I0) IC28.5(B:I0) IC28.8(C:I0) IC28.12(D:I0)
N$20: IC15.10(C:O) IC18.1(A:I0) IC18.5(B:I0) IC18.8(C:I0) IC18.12(D:I0)
N$21: IC19.4(B:O) IC20.3(A:CLK) IC20.13(B:CLK) IC21.3(A:CLK) IC21.13(B:CLK)
N$22: IC10.1(A:Q) IC14.2(A:I1) JP16.1
N$23: IC11.15(B:Q) IC14.13(D:I1) JP19.1
N$24: IC11.1(A:Q) IC14.9(C:I1) JP18.1
N$25: IC10.15(B:Q) IC14.6(B:I1) JP17.1
N$27: IC19.3(A:O) IC23.1(A:I0) IC23.5(B:I0) IC23.8(C:I0) IC23.12(D:I0)
N$28: IC27.10(C:O) IC68.1(A:I0) IC68.5(B:I0) IC68.8(C:I0) IC68.12(D:I0)
N$29: IC31.11(B:K) IC114.6(C:O)
N$30: IC27.3(A:O) IC63.1(A:I0) IC63.5(B:I0) IC63.8(C:I0) IC63.12(D:I0)
N$31: IC31.5(A:K) IC114.10(D:O)
N$32: IC16.11(B:K) IC116.6(C:O)
N$33: IC16.5(A:K) IC116.10(D:O)
N$34: IC12.11(B:K) IC116.12(E:O)
N$35: IC12.5(A:K) IC116.15(F:O)
N$36: IC10.3(A:CLK) IC10.13(B:CLK) IC11.3(A:CLK) IC11.13(B:CLK) IC15.4(B:O)
N$37: IC32.11(D:O) IC85.3(A:CLK) IC85.13(B:CLK) IC86.3(A:CLK) IC86.13(B:CLK)
N$38: IC32.4(B:O) IC80.3(A:CLK) IC80.13(B:CLK) IC81.3(A:CLK) IC81.13(B:CLK)
N$39: IC29.11(D:O) IC75.3(A:CLK) IC75.13(B:CLK) IC76.3(A:CLK) IC76.13(B:CLK)
N$40: IC12.1(A:Q) IC18.2(A:I1)
N$41: IC16.15(B:Q) IC18.13(D:I1)
N$42: IC16.1(A:Q) IC18.9(C:I1)
N$43: IC12.15(B:Q) IC18.6(B:I1)
N$45: IC30.11(B:K) IC114.12(E:O)
N$46: IC30.5(A:K) IC114.15(F:O)
N$47: IC19.11(D:O) IC25.3(A:CLK) IC25.13(B:CLK) IC26.3(A:CLK) IC26.13(B:CLK)
N$48: IC13.4(B:O) IC30.3(A:CLK) IC30.13(B:CLK) IC31.3(A:CLK) IC31.13(B:CLK)
N$49: IC24.10(C:O) IC58.1(A:I0) IC58.5(B:I0) IC58.8(C:I0) IC58.12(D:I0)
N$50: IC21.11(B:K) IC115.12(E:O)
N$51: IC21.5(A:K) IC115.15(F:O)
N$52: IC20.11(B:K) IC116.2(A:O)
N$53: IC20.5(A:K) IC116.4(B:O)
N$54: IC13.3(A:O) IC33.1(A:I0) IC33.5(B:I0) IC33.8(C:I0) IC33.12(D:I0)
N$55: IC13.10(C:O) IC38.1(A:I0) IC38.5(B:I0) IC38.8(C:I0) IC38.12(D:I0)
N$56: IC17.3(A:O) IC43.1(A:I0) IC43.5(B:I0) IC43.8(C:I0) IC43.12(D:I0)
N$57: IC13.11(D:O) IC35.3(A:CLK) IC35.13(B:CLK) IC36.3(A:CLK) IC36.13(B:CLK)
N$58: IC20.1(A:Q) IC23.2(A:I1)
N$59: IC21.15(B:Q) IC23.13(D:I1)
N$60: IC21.1(A:Q) IC23.9(C:I1)
N$61: IC20.15(B:Q) IC23.6(B:I1)
N$63: IC24.3(A:O) IC53.1(A:I0) IC53.5(B:I0) IC53.8(C:I0) IC53.12(D:I0)
N$64: IC17.11(D:O) IC45.3(A:CLK) IC45.13(B:CLK) IC46.3(A:CLK) IC46.13(B:CLK)
N$65: IC26.11(B:K) IC115.2(A:O)
N$66: IC26.5(A:K) IC115.4(B:O)
N$67: IC25.11(B:K) IC115.6(C:O)
N$68: IC25.5(A:K) IC115.10(D:O)
N$69: IC17.4(B:O) IC40.3(A:CLK) IC40.13(B:CLK) IC41.3(A:CLK) IC41.13(B:CLK)
N$70: IC17.10(C:O) IC48.1(A:I0) IC48.5(B:I0) IC48.8(C:I0) IC48.12(D:I0)
N$71: CLK.1 IC34.2(A:I1)
N$72: IC34.1(A:I0) W.1
N$73: IC25.1(A:Q) IC28.2(A:I1)
N$74: IC26.15(B:Q) IC28.13(D:I1)
N$75: IC26.1(A:Q) IC28.9(C:I1)
N$76: IC25.15(B:Q) IC28.6(B:I1)
N$83: IC30.1(A:Q) IC33.2(A:I1)
N$84: IC31.15(B:Q) IC33.13(D:I1)
N$85: IC31.1(A:Q) IC33.9(C:I1)
N$86: IC30.15(B:Q) IC33.6(B:I1)
N$90: IC36.11(B:K) IC113.12(E:O)
N$91: IC36.5(A:K) IC113.15(F:O)
N$92: IC35.11(B:K) IC114.2(A:O)
N$93: IC35.5(A:K) IC114.4(B:O)
N$98: IC35.1(A:Q) IC38.2(A:I1)
N$99: IC36.15(B:Q) IC38.13(D:I1)
N$100: IC36.1(A:Q) IC38.9(C:I1)
N$101: IC35.15(B:Q) IC38.6(B:I1)
N$103: IC29.4(B:O) IC70.3(A:CLK) IC70.13(B:CLK) IC71.3(A:CLK) IC71.13(B:CLK)
N$104: IC41.11(B:K) IC113.2(A:O)
N$105: IC41.5(A:K) IC113.4(B:O)
N$106: IC40.11(B:K) IC113.6(C:O)
N$107: IC40.5(A:K) IC113.10(D:O)
N$112: IC40.1(A:Q) IC43.2(A:I1)
N$113: IC41.15(B:Q) IC43.13(D:I1)
N$114: IC41.1(A:Q) IC43.9(C:I1)
N$115: IC40.15(B:Q) IC43.6(B:I1)
N$118: IC24.4(B:O) IC50.3(A:CLK) IC50.13(B:CLK) IC51.3(A:CLK) IC51.13(B:CLK)
N$119: IC46.11(B:K) IC112.6(C:O)
N$120: IC46.5(A:K) IC112.10(D:O)
N$121: IC45.11(B:K) IC112.12(E:O)
N$122: IC45.5(A:K) IC112.15(F:O)
N$127: IC45.1(A:Q) IC48.2(A:I1)
N$128: IC46.15(B:Q) IC48.13(D:I1)
N$129: IC46.1(A:Q) IC48.9(C:I1)
N$130: IC45.15(B:Q) IC48.6(B:I1)
N$132: IC51.11(B:K) IC111.12(E:O)
N$134: IC51.5(A:K) IC111.15(F:O)
N$135: IC50.11(B:K) IC112.2(A:O)
N$136: IC50.5(A:K) IC112.4(B:O)
N$141: IC50.1(A:Q) IC53.2(A:I1)
N$142: IC51.15(B:Q) IC53.13(D:I1)
N$143: IC51.1(A:Q) IC53.9(C:I1)
N$144: IC50.15(B:Q) IC53.6(B:I1)
N$147: IC27.11(D:O) IC65.3(A:CLK) IC65.13(B:CLK) IC66.3(A:CLK) IC66.13(B:CLK)
N$148: IC56.11(B:K) IC111.2(A:O)
N$149: IC56.5(A:K) IC111.4(B:O)
N$150: IC55.11(B:K) IC111.6(C:O)
N$151: IC55.5(A:K) IC111.10(D:O)
N$156: IC55.1(A:Q) IC58.2(A:I1)
N$157: IC56.15(B:Q) IC58.13(D:I1)
N$158: IC56.1(A:Q) IC58.9(C:I1)
N$159: IC55.15(B:Q) IC58.6(B:I1)
N$161: IC27.4(B:O) IC60.3(A:CLK) IC60.13(B:CLK) IC61.3(A:CLK) IC61.13(B:CLK)
N$162: IC61.11(B:K) IC110.6(C:O)
N$163: IC61.5(A:K) IC110.10(D:O)
N$164: IC60.11(B:K) IC110.12(E:O)
N$165: IC60.5(A:K) IC110.15(F:O)
N$170: IC60.1(A:Q) IC63.2(A:I1)
N$171: IC61.15(B:Q) IC63.13(D:I1)
N$172: IC61.1(A:Q) IC63.9(C:I1)
N$173: IC60.15(B:Q) IC63.6(B:I1)
N$175: IC24.11(D:O) IC55.3(A:CLK) IC55.13(B:CLK) IC56.3(A:CLK) IC56.13(B:CLK)
N$177: IC66.11(B:K) IC109.12(E:O)
N$178: IC66.5(A:K) IC109.15(F:O)
N$179: IC65.11(B:K) IC110.2(A:O)
N$180: IC65.5(A:K) IC110.4(B:O)
N$185: IC65.1(A:Q) IC68.2(A:I1)
N$186: IC66.15(B:Q) IC68.13(D:I1)
N$187: IC66.1(A:Q) IC68.9(C:I1)
N$188: IC65.15(B:Q) IC68.6(B:I1)
N$194: IC71.11(B:K) IC109.2(A:O)
N$195: IC71.5(A:K) IC109.4(B:O)
N$196: IC70.11(B:K) IC109.6(C:O)
N$197: IC70.5(A:K) IC109.10(D:O)
N$202: IC70.1(A:Q) IC73.2(A:I1)
N$203: IC71.15(B:Q) IC73.13(D:I1)
N$204: IC71.1(A:Q) IC73.9(C:I1)
N$205: IC70.15(B:Q) IC73.6(B:I1)
N$208: IC76.11(B:K) IC108.6(C:O)
N$209: IC76.5(A:K) IC108.10(D:O)
N$210: IC75.11(B:K) IC108.12(E:O)
N$211: IC75.5(A:K) IC108.15(F:O)
N$216: IC75.1(A:Q) IC78.2(A:I1)
N$217: IC76.15(B:Q) IC78.13(D:I1)
N$218: IC76.1(A:Q) IC78.9(C:I1)
N$219: IC75.15(B:Q) IC78.6(B:I1)
N$222: IC22.15(F:O) IC81.11(B:K)
N$223: IC81.5(A:K) IC108.2(A:O)
N$224: IC22.10(D:O) IC80.11(B:K)
N$225: IC80.5(A:K) IC108.4(B:O)
N$230: IC80.1(A:Q) IC83.2(A:I1)
N$231: IC81.15(B:Q) IC83.13(D:I1)
N$232: IC81.1(A:Q) IC83.9(C:I1)
N$233: IC80.15(B:Q) IC83.6(B:I1)
N$237: IC22.2(A:O) IC86.11(B:K)
N$238: IC22.4(B:O) IC86.5(A:K)
N$239: IC22.6(C:O) IC85.11(B:K)
N$240: IC22.12(E:O) IC85.5(A:K)
N$245: IC85.1(A:Q) IC88.2(A:I1)
N$246: IC86.15(B:Q) IC88.13(D:I1)
N$247: IC86.1(A:Q) IC88.9(C:I1)
N$248: IC85.15(B:Q) IC88.6(B:I1)
NUMBER1: IC10.6(A:J) IC12.6(A:J) IC20.6(A:J) IC22.11(E:I) IC25.6(A:J) IC30.6(A:J) IC35.6(A:J) IC40.6(A:J) IC45.6(A:J) IC50.6(A:J) IC55.6(A:J) IC60.6(A:J) IC65.6(A:J) IC70.6(A:J) IC75.6(A:J) IC80.6(A:J) IC85.6(A:J) IC108.5(B:I) IC108.14(F:I) IC109.9(D:I) IC110.5(B:I) IC110.14(F:I) IC111.9(D:I) IC112.5(B:I) IC112.14(F:I) IC113.9(D:I) IC114.5(B:I) IC114.14(F:I) IC115.9(D:I) IC116.5(B:I) IC116.14(F:I) IC117.9(D:I) NUMBER.1
NUMBER2: IC10.10(B:J) IC12.10(B:J) IC20.10(B:J) IC22.7(C:I) IC22.9(D:I) IC25.10(B:J) IC30.10(B:J) IC35.10(B:J) IC40.10(B:J) IC45.10(B:J) IC50.10(B:J) IC55.10(B:J) IC60.10(B:J) IC65.10(B:J) IC70.10(B:J) IC75.10(B:J) IC80.10(B:J) IC85.10(B:J) IC108.11(E:I) IC109.7(C:I) IC110.3(A:I) IC110.11(E:I) IC111.7(C:I) IC112.3(A:I) IC112.11(E:I) IC113.7(C:I) IC114.3(A:I) IC114.11(E:I) IC115.7(C:I) IC116.3(A:I) IC116.11(E:I) IC117.7(C:I) NUMBER.2
NUMBER3: IC11.6(A:J) IC16.6(A:J) IC21.6(A:J) IC22.5(B:I) IC26.6(A:J) IC31.6(A:J) IC36.6(A:J) IC41.6(A:J) IC46.6(A:J) IC51.6(A:J) IC56.6(A:J) IC61.6(A:J) IC66.6(A:J) IC71.6(A:J) IC76.6(A:J) IC81.6(A:J) IC86.6(A:J) IC108.3(A:I) IC108.9(D:I) IC109.5(B:I) IC109.14(F:I) IC110.9(D:I) IC111.5(B:I) IC111.14(F:I) IC112.9(D:I) IC113.5(B:I) IC113.14(F:I) IC114.9(D:I) IC115.5(B:I) IC115.14(F:I) IC116.9(D:I) IC117.5(B:I) NUMBER.3
NUMBER4: IC11.10(B:J) IC16.10(B:J) IC21.10(B:J) IC22.3(A:I) IC22.14(F:I) IC26.10(B:J) IC31.10(B:J) IC36.10(B:J) IC41.10(B:J) IC46.10(B:J) IC51.10(B:J) IC56.10(B:J) IC61.10(B:J) IC66.10(B:J) IC71.10(B:J) IC76.10(B:J) IC81.10(B:J) IC86.10(B:J) IC108.7(C:I) IC109.3(A:I) IC109.11(E:I) IC110.7(C:I) IC111.3(A:I) IC111.11(E:I) IC112.7(C:I) IC113.3(A:I) IC113.11(E:I) IC114.7(C:I) IC115.3(A:I) IC115.11(E:I) IC116.7(C:I) IC117.3(A:I) NUMBER.4
O0: IC83.3(A:O) ; also sheet 3
O1: IC83.4(B:O) ; also sheet 3
O2: IC83.10(C:O) ; also sheet 3
O3: IC83.11(D:O) ; also sheet 3
P0: IC88.3(A:O) ; also sheet 3
P1: IC88.4(B:O) ; also sheet 3
P2: IC88.10(C:O) ; also sheet 3
P3: IC88.11(D:O) ; also sheet 3
R: IC13.1(A:I0) IC13.8(C:I0) IC15.1(A:I0) IC15.8(C:I0) IC17.1(A:I0) IC17.8(C:I0) IC19.1(A:I0) IC19.8(C:I0) IC24.1(A:I0) IC24.8(C:I0) IC27.1(A:I0) IC27.8(C:I0) IC29.1(A:I0) IC29.8(C:I0) IC32.1(A:I0) IC32.8(C:I0) R.1
W: IC13.5(B:I0) IC13.12(D:I0) IC15.5(B:I0) IC15.12(D:I0) IC17.5(B:I0) IC17.12(D:I0) IC19.5(B:I0) IC19.12(D:I0) IC24.5(B:I0) IC24.12(D:I0) IC27.5(B:I0) IC27.12(D:I0) IC29.5(B:I0) IC29.12(D:I0) IC32.5(B:I0) IC32.12(D:I0) IC34.3(A:O)
Unconnected: IC10.2(A:!Q) IC10.14(B:!Q) IC11.2(A:!Q) IC11.14(B:!Q) IC12.2(A:!Q) IC12.14(B:!Q) IC16.2(A:!Q) IC16.14(B:!Q) IC20.2(A:!Q) IC20.14(B:!Q) IC21.2(A:!Q) IC21.14(B:!Q) IC25.2(A:!Q) IC25.14(B:!Q) IC26.2(A:!Q) IC26.14(B:!Q) IC30.2(A:!Q) IC30.14(B:!Q) IC31.2(A:!Q) IC31.14(B:!Q) IC34.4(B:O) IC34.10(C:O) IC34.11(D:O) IC35.2(A:!Q) IC35.14(B:!Q) IC36.2(A:!Q) IC36.14(B:!Q) IC40.2(A:!Q) IC40.14(B:!Q) IC41.2(A:!Q) IC41.14(B:!Q) IC45.2(A:!Q) IC45.14(B:!Q) IC46.2(A:!Q) IC46.14(B:!Q) IC50.2(A:!Q) IC50.14(B:!Q) IC51.2(A:!Q) IC51.14(B:!Q) IC55.2(A:!Q) IC55.14(B:!Q) IC56.2(A:!Q) IC56.14(B:!Q) IC60.2(A:!Q) IC60.14(B:!Q) IC61.2(A:!Q) IC61.14(B:!Q) IC65.2(A:!Q) IC65.14(B:!Q) IC66.2(A:!Q) IC66.14(B:!Q) IC70.2(A:!Q) IC70.14(B:!Q) IC71.2(A:!Q) IC71.14(B:!Q) IC75.2(A:!Q) IC75.14(B:!Q) IC76.2(A:!Q) IC76.14(B:!Q) IC80.2(A:!Q) IC80.14(B:!Q) IC81.2(A:!Q) IC81.14(B:!Q) IC85.2(A:!Q) IC85.14(B:!Q) IC86.2(A:!Q) IC86.14(B:!Q) IC117.12(E:O) IC117.15(F:O)

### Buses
A[0..3],B[0..3],C[0..3],D[0..3],E[0..3],F[0..3],G[0..3],H[0..3],I[0..3],J[0..3],K[0..3],L[0..3],M[0..3],N[0..3],O[0..3],P[0..3]

## Sheet 3 of 3: Register Output
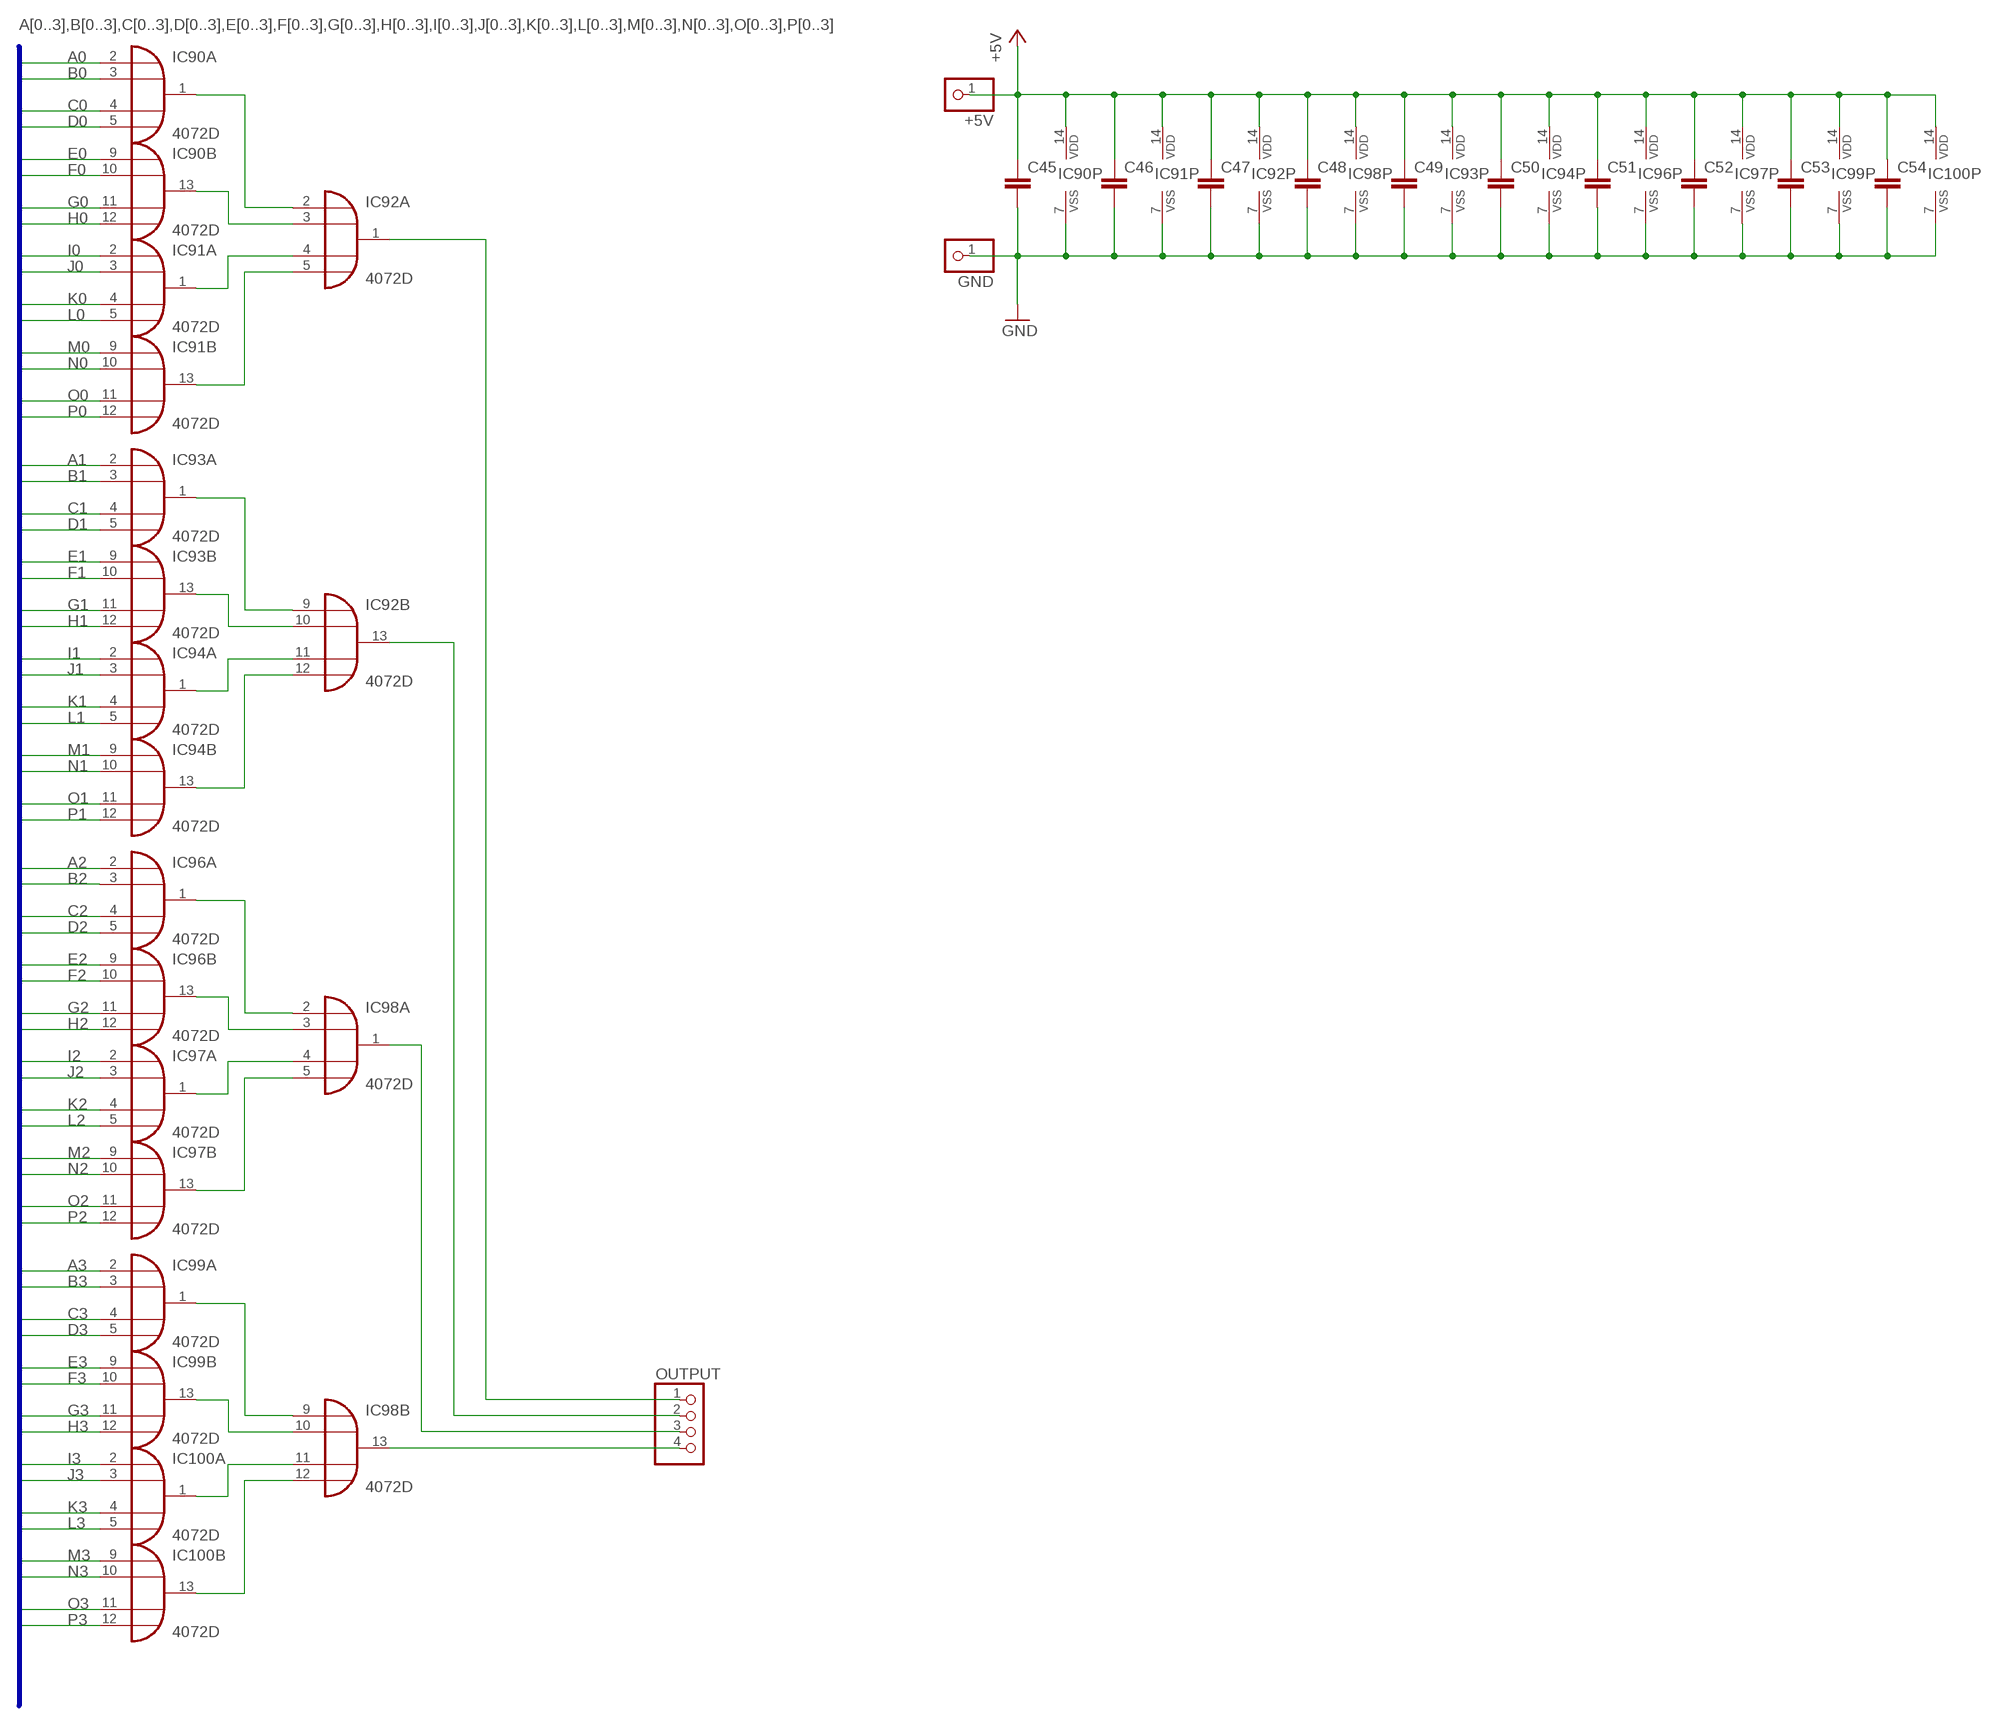
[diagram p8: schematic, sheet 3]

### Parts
+5V  PINHD-1X1  [1X01]
C45  C-EUC0805  [C0805]
C46  C-EUC0805  [C0805]
C47  C-EUC0805  [C0805]
C48  C-EUC0805  [C0805]
C49  C-EUC0805  [C0805]
C50  C-EUC0805  [C0805]
C51  C-EUC0805  [C0805]
C52  C-EUC0805  [C0805]
C53  C-EUC0805  [C0805]
C54  C-EUC0805  [C0805]
GND  PINHD-1X1  [1X01]
IC90  4072D  [SO14]
IC91  4072D  [SO14]
IC92  4072D  [SO14]
IC93  4072D  [SO14]
IC94  4072D  [SO14]
IC96  4072D  [SO14]
IC97  4072D  [SO14]
IC98  4072D  [SO14]
IC99  4072D  [SO14]
IC100  4072D  [SO14]
OUTPUT  PINHD-1X4  [1X04]

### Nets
+5V: +5V.1 C45.1 C46.1 C47.1 C48.1 C49.1 C50.1 C51.1 C52.1 C53.1 C54.1 IC90.14(P:VDD) IC91.14(P:VDD) IC92.14(P:VDD) IC93.14(P:VDD) IC94.14(P:VDD) IC96.14(P:VDD) IC97.14(P:VDD) IC98.14(P:VDD) IC99.14(P:VDD) IC100.14(P:VDD) ; also sheet 1,2
A0: IC90.2(A:I0) ; also sheet 2
A1: IC93.2(A:I0) ; also sheet 2
A2: IC96.2(A:I0) ; also sheet 2
A3: IC99.2(A:I0) ; also sheet 2
B0: IC90.3(A:I1) ; also sheet 2
B1: IC93.3(A:I1) ; also sheet 2
B2: IC96.3(A:I1) ; also sheet 2
B3: IC99.3(A:I1) ; also sheet 2
C0: IC90.4(A:I2) ; also sheet 2
C1: IC93.4(A:I2) ; also sheet 2
C2: IC96.4(A:I2) ; also sheet 2
C3: IC99.4(A:I2) ; also sheet 2
D0: IC90.5(A:I3) ; also sheet 2
D1: IC93.5(A:I3) ; also sheet 2
D2: IC96.5(A:I3) ; also sheet 2
D3: IC99.5(A:I3) ; also sheet 2
E0: IC90.9(B:I0) ; also sheet 2
E1: IC93.9(B:I0) ; also sheet 2
E2: IC96.9(B:I0) ; also sheet 2
E3: IC99.9(B:I0) ; also sheet 2
F0: IC90.10(B:I1) ; also sheet 2
F1: IC93.10(B:I1) ; also sheet 2
F2: IC96.10(B:I1) ; also sheet 2
F3: IC99.10(B:I1) ; also sheet 2
G0: IC90.11(B:I2) ; also sheet 2
G1: IC93.11(B:I2) ; also sheet 2
G2: IC96.11(B:I2) ; also sheet 2
G3: IC99.11(B:I2) ; also sheet 2
GND: C45.2 C46.2 C47.2 C48.2 C49.2 C50.2 C51.2 C52.2 C53.2 C54.2 GND.1 IC90.7(P:VSS) IC91.7(P:VSS) IC92.7(P:VSS) IC93.7(P:VSS) IC94.7(P:VSS) IC96.7(P:VSS) IC97.7(P:VSS) IC98.7(P:VSS) IC99.7(P:VSS) IC100.7(P:VSS) ; also sheet 1,2
H0: IC90.12(B:I3) ; also sheet 2
H1: IC93.12(B:I3) ; also sheet 2
H2: IC96.12(B:I3) ; also sheet 2
H3: IC99.12(B:I3) ; also sheet 2
I0: IC91.2(A:I0) ; also sheet 2
I1: IC94.2(A:I0) ; also sheet 2
I2: IC97.2(A:I0) ; also sheet 2
I3: IC100.2(A:I0) ; also sheet 2
J0: IC91.3(A:I1) ; also sheet 2
J1: IC94.3(A:I1) ; also sheet 2
J2: IC97.3(A:I1) ; also sheet 2
J3: IC100.3(A:I1) ; also sheet 2
K0: IC91.4(A:I2) ; also sheet 2
K1: IC94.4(A:I2) ; also sheet 2
K2: IC97.4(A:I2) ; also sheet 2
K3: IC100.4(A:I2) ; also sheet 2
L0: IC91.5(A:I3) ; also sheet 2
L1: IC94.5(A:I3) ; also sheet 2
L2: IC97.5(A:I3) ; also sheet 2
L3: IC100.5(A:I3) ; also sheet 2
M0: IC91.9(B:I0) ; also sheet 2
M1: IC94.9(B:I0) ; also sheet 2
M2: IC97.9(B:I0) ; also sheet 2
M3: IC100.9(B:I0) ; also sheet 2
N0: IC91.10(B:I1) ; also sheet 2
N1: IC94.10(B:I1) ; also sheet 2
N2: IC97.10(B:I1) ; also sheet 2
N3: IC100.10(B:I1) ; also sheet 2
N$26: IC90.1(A:O) IC92.2(A:I0)
N$44: IC96.1(A:O) IC98.2(A:I0)
N$62: IC90.13(B:O) IC92.3(A:I1)
N$77: IC91.1(A:O) IC92.4(A:I2)
N$87: IC91.13(B:O) IC92.5(A:I3)
N$102: IC92.9(B:I0) IC93.1(A:O)
N$116: IC92.10(B:I1) IC93.13(B:O)
N$131: IC92.11(B:I2) IC94.1(A:O)
N$133: IC92.12(B:I3) IC94.13(B:O)
N$145: IC96.13(B:O) IC98.3(A:I1)
N$146: IC97.1(A:O) IC98.4(A:I2)
N$160: IC97.13(B:O) IC98.5(A:I3)
N$174: IC98.9(B:I0) IC99.1(A:O)
N$189: IC98.10(B:I1) IC99.13(B:O)
N$190: IC98.11(B:I2) IC100.1(A:O)
N$191: IC98.12(B:I3) IC100.13(B:O)
N$192: IC98.13(B:O) OUTPUT.4
N$206: IC98.1(A:O) OUTPUT.3
N$220: IC92.13(B:O) OUTPUT.2
N$234: IC92.1(A:O) OUTPUT.1
O0: IC91.11(B:I2) ; also sheet 2
O1: IC94.11(B:I2) ; also sheet 2
O2: IC97.11(B:I2) ; also sheet 2
O3: IC100.11(B:I2) ; also sheet 2
P0: IC91.12(B:I3) ; also sheet 2
P1: IC94.12(B:I3) ; also sheet 2
P2: IC97.12(B:I3) ; also sheet 2
P3: IC100.12(B:I3) ; also sheet 2

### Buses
A[0..3],B[0..3],C[0..3],D[0..3],E[0..3],F[0..3],G[0..3],H[0..3],I[0..3],J[0..3],K[0..3],L[0..3],M[0..3],N[0..3],O[0..3],P[0..3]

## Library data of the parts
+5V CLK GND JP16-JP19 R W = pinhead:PINHD-1X1: PIN HEADER
ADRESS NUMBER OUTPUT = pinhead:PINHD-1X4: PIN HEADER
C1-C87 = rcl:C-EU: CAPACITOR, European symbol; SPICEPREFIX: C
IC1-IC8 = 40xx:4082: Dual 4-input AND
IC9 IC22 IC108-IC117 = 40xx:4049: Hex inverting BUFFER
IC10-IC12 IC16 IC20 IC21 IC25 IC26 IC30 IC31 IC35 IC36 IC40 IC41 IC45 IC46 IC50 IC51 IC55 IC56 IC60 IC61 IC65 IC66 IC70 IC71 IC75 IC76 IC80 IC81 IC85 IC86 = 40xx:4027: Dual JK FLIP FLOP
IC13-IC15 IC17-IC19 IC23 IC24 IC27-IC29 IC32-IC34 IC38 IC43 IC48 IC53 IC58 IC63 IC68 IC73 IC78 IC83 IC88 = 40xx:4081: Quad 2-input AND
IC90-IC94 IC96-IC100 = 40xx:4072: Dual 4-input OR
